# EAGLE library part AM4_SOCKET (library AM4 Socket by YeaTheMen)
Single Piece AM4 Socket Symbol. Every single one of the 1331 pins here in order Yours truly, YeaTheMen
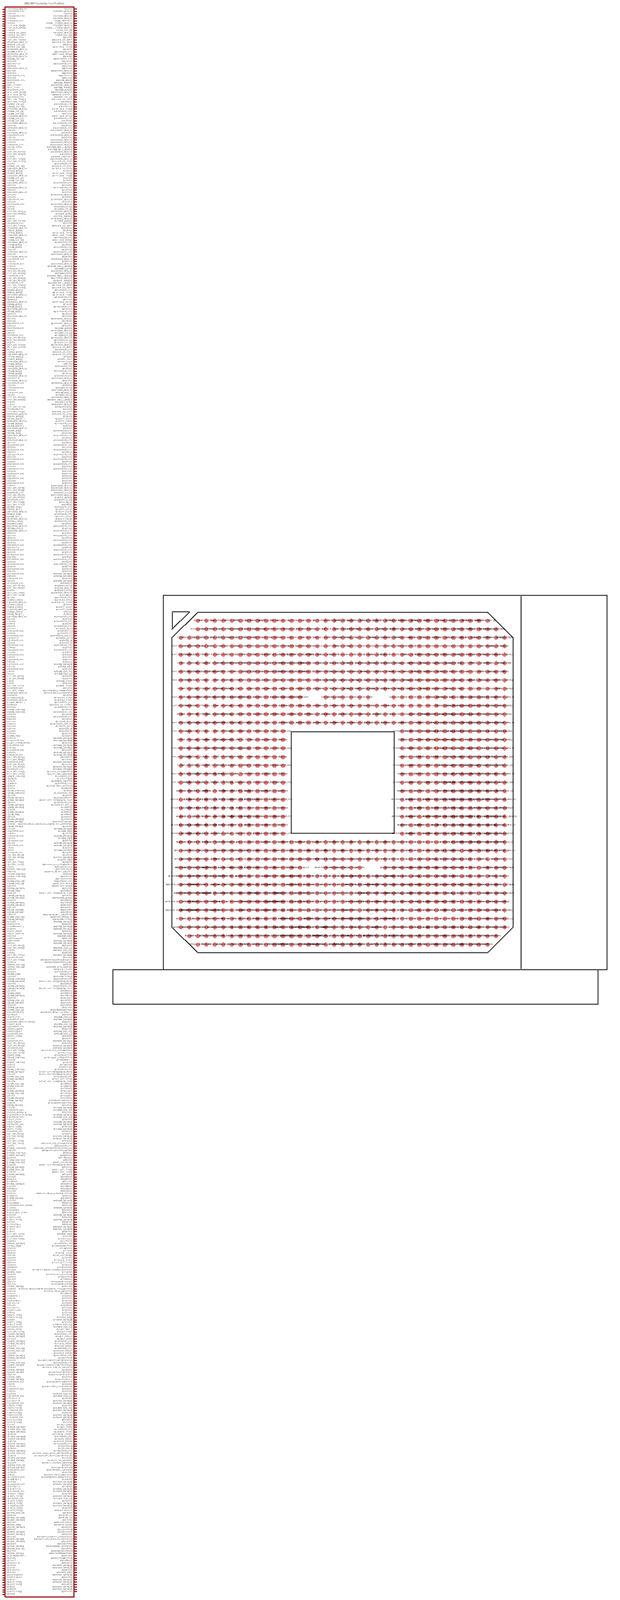
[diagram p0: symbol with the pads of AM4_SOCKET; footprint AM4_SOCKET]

Designator prefix -

## AM4_SOCKET  [AM4_SOCKET]
A3.VSS  A3.VSS  out
A4.DP0_TXN[2]  A4.DP0_TXN[2]
A5.RSVD  A5.RSVD  nc
A6.VSS  A6.VSS  out
A7.DP2_TXP[1]  A7.DP2_TXP[1]
A8.DP2_TXN[1]  A8.DP2_TXN[1]
A9.VSS  A9.VSS  out
A10.DP2_AUXP  A10.DP2_AUXP
A11.DP2_AUXN  A11.DP2_AUXN
A12.VSS  A12.VSS  out
A13.TEST11  A13.TEST11
A14.TDI  A14.TDI
A15.VSS  A15.VSS  out
A16.TEST41  A16.TEST41
A17.SVT  A17.SVT
A18.VSS  A18.VSS  out
A19.THERMTRIP_L  A19.THERMTRIP_L
A20.MB_DATA[4]  A20.MB_DATA[4]
A21.VSS  A21.VSS  out
A22.MB_DQS_L[0]  A22.MB_DQS_L[0]
A23.MB_DATA[6]  A23.MB_DATA[6]
A24.VSS  A24.VSS  out
A25.MB_DATA[12]  A25.MB_DATA[12]
A26.MB_DATA[8]  A26.MB_DATA[8]
A27.VSS  A27.VSS  out
A28.MB_DATA[14]  A28.MB_DATA[14]
A29.MB_DATA[10]  A29.MB_DATA[10]
A30.VSS  A30.VSS  out
A31.MB_DATA[16]  A31.MB_DATA[16]
A32.MB_DM[2]  A32.MB_DM[2]
A33.VSS  A33.VSS  out
A34.MB_DATA[23]  A34.MB_DATA[23]
A35.MB_DATA[28]  A35.MB_DATA[28]
A36.VSS  A36.VSS  out
A37.MB_DQS_L[3]  A37.MB_DQS_L[3]
AA1.VSS  AA1.VSS  out
AA2.USB_SS_1RXP  AA2.USB_SS_1RXP
AA3.USB_SS_1RXN  AA3.USB_SS_1RXN
AA4.VSS  AA4.VSS  out
AA5.P_HUB_TXP[1]  AA5.P_HUB_TXP[1]
AA6.VSS  AA6.VSS  out
AA7.VDDCR_CPU  AA7.VDDCR_CPU  pwr
AA8.P_HUB_RXN[1]  AA8.P_HUB_RXN[1]
AA9.VSS  AA9.VSS  out
AA10.VDDCR_CPU  AA10.VDDCR_CPU  pwr
AA11.VSS  AA11.VSS  out
AA12.VDDCR_CPU  AA12.VDDCR_CPU  pwr
AA13.VSS  AA13.VSS  out
AA27.VSS  AA27.VSS  out
AA28.VDDIO_MEM_S3  AA28.VDDIO_MEM_S3  pwr
AA29.VSS  AA29.VSS  out
AA30.TEST31  AA30.TEST31
AA31.VSS  AA31.VSS  out
AA32.MA_ADD[0]  AA32.MA_ADD[0]
AA33.MA_BANK[1]  AA33.MA_BANK[1]
AA34.VDDIO_MEM_S3  AA34.VDDIO_MEM_S3  pwr
AA35.MA_BANK[0]  AA35.MA_BANK[0]
AA36.MA_ADD[10]  AA36.MA_ADD[10]
AA37.VDDIO_MEM_S3  AA37.VDDIO_MEM_S3  pwr
AA38.MB_EVENT_L  AA38.MB_EVENT_L
AA39.MB_CLK_L[3]  AA39.MB_CLK_L[3]
AB1.USB_SS_1TXP  AB1.USB_SS_1TXP
AB2.RSVD  AB2.RSVD  nc
AB3.VDDCR_CPU  AB3.VDDCR_CPU  pwr
AB4.TEST10  AB4.TEST10
AB5.P_HUB_TXN[1]  AB5.P_HUB_TXN[1]
AB6.VDDCR_CPU  AB6.VDDCR_CPU  pwr
AB7.VSS  AB7.VSS  out
AB8.P_HUB_RXP[1]  AB8.P_HUB_RXP[1]
AB9.VDDCR_CPU  AB9.VDDCR_CPU  pwr
AB10.VSS  AB10.VSS  out
AB11.VDDCR_CPU  AB11.VDDCR_CPU  pwr
AB12.VSS  AB12.VSS  out
AB13.VDDCR_CPU  AB13.VDDCR_CPU  pwr
AB27.VDDIO_MEM_S3  AB27.VDDIO_MEM_S3  pwr
AB28.VSS  AB28.VSS  out
AB29.VDDIO_MEM_S3  AB29.VDDIO_MEM_S3  pwr
AB30.VSS  AB30.VSS  out
AB31.VDDIO_MEM_S3  AB31.VDDIO_MEM_S3  pwr
AB32.VDDIO_MEM_S3  AB32.VDDIO_MEM_S3  pwr
AB33.VDDIO_MEM_S3  AB33.VDDIO_MEM_S3  pwr
AB34.MA_RAS_L_ADD[16]  AB34.MA_RAS_L_ADD[16]
AB35.MA_WE_L_ADD[14]  AB35.MA_WE_L_ADD[14]
AB36.VDDIO_MEM_S3  AB36.VDDIO_MEM_S3  pwr
AB37.RSVD  AB37.RSVD  nc
AB38.MB_PARTOUT  AB38.MB_PARTOUT  out
AB39.VDDIO_MEM_S3  AB39.VDDIO_MEM_S3  pwr
AC1.USB_SS_1TXN  AC1.USB_SS_1TXN
AC2.VDDCR_CPU  AC2.VDDCR_CPU  pwr
AC3.USB_SS_2TXP  AC3.USB_SS_2TXP
AC4.USB_SS_2TXN  AC4.USB_SS_2TXN
AC5.VSS  AC5.VSS  out
AC6.P_HUB_TXP[2]  AC6.P_HUB_TXP[2]
AC7.P_HUB_TXN[2]  AC7.P_HUB_TXN[2]
AC8.VSS  AC8.VSS  out
AC9.VSS  AC9.VSS  out
AC10.VDDCR_CPU  AC10.VDDCR_CPU  pwr
AC11.VSS  AC11.VSS  out
AC12.VDDCR_CPU  AC12.VDDCR_CPU  pwr
AC13.VSS  AC13.VSS  out
AC27.VSS  AC27.VSS  out
AC28.VDDIO_MEM_S3  AC28.VDDIO_MEM_S3  pwr
AC29.VSS  AC29.VSS  out
AC30.VDDIO_MEM_S3  AC30.VDDIO_MEM_S3  pwr
AC31.VSS  AC31.VSS  out
AC32.VDDIO_MEM_S3  AC32.VDDIO_MEM_S3  pwr
AC33.MA0_CS_L[0]  AC33.MA0_CS_L[0]
AC34.MA1_CS_L[0]  AC34.MA1_CS_L[0]
AC35.VDDIO_MEM_S3  AC35.VDDIO_MEM_S3  pwr
AC36.MB_ADD[0]  AC36.MB_ADD[0]
AC37.MB_BANK[1]  AC37.MB_BANK[1]
AC38.VDDIO_MEM_S3  AC38.VDDIO_MEM_S3  pwr
AC39.MB_ADD[10]  AC39.MB_ADD[10]
AD1.VSS  AD1.VSS  out
AD2.USB_SS_3RXP  AD2.USB_SS_3RXP
AD3.RSVD  AD3.RSVD  nc
AD4.VSS  AD4.VSS  out
AD5.P_HUB_TXP[3]  AD5.P_HUB_TXP[3]
AD6.P_HUB_TXN[3]  AD6.P_HUB_TXN[3]
AD7.VDDCR_CPU  AD7.VDDCR_CPU  pwr
AD8.P_HUB_RXN[0]  AD8.P_HUB_RXN[0]
AD9.VDDCR_CPU  AD9.VDDCR_CPU  pwr
AD10.VSS  AD10.VSS  out
AD11.VDDCR_CPU  AD11.VDDCR_CPU  pwr
AD12.VSS  AD12.VSS  out
AD13.VDDCR_CPU  AD13.VDDCR_CPU  pwr
AD27.VDDIO_MEM_S3  AD27.VDDIO_MEM_S3  pwr
AD28.VSS  AD28.VSS  out
AD29.VDDIO_MEM_S3  AD29.VDDIO_MEM_S3  pwr
AD30.VSS  AD30.VSS  out
AD31.VDDIO_MEM_S3  AD31.VDDIO_MEM_S3  pwr
AD32.MA_CAS_L_ADD[15]  AD32.MA_CAS_L_ADD[15]
AD33.MA1_ODT[0]  AD33.MA1_ODT[0]
AD34.VDDIO_MEM_S3  AD34.VDDIO_MEM_S3  pwr
AD35.MA0_ODT[0]  AD35.MA0_ODT[0]
AD36.MB_RAS_L_ADD[16]  AD36.MB_RAS_L_ADD[16]
AD37.VDDIO_MEM_S3  AD37.VDDIO_MEM_S3  pwr
AD38.MB_BANK[0]  AD38.MB_BANK[0]
AD39.MB_WE_L_ADD[14]  AD39.MB_WE_L_ADD[14]
AE1.USB_SS_3RXP  AE1.USB_SS_3RXP
AE2.USB_SS_2RXN  AE2.USB_SS_2RXN
AE3.VDDCR_CPU  AE3.VDDCR_CPU  pwr
AE4.P_HUB_TXP[0]  AE4.P_HUB_TXP[0]
AE5.P_HUB_TXN[0]  AE5.P_HUB_TXN[0]
AE6.VDDCR_CPU  AE6.VDDCR_CPU  pwr
AE7.VSS  AE7.VSS  out
AE8.P_HUB_RXP[0]  AE8.P_HUB_RXP[0]
AE9.VSS  AE9.VSS  out
AE10.VDDCR_CPU  AE10.VDDCR_CPU  pwr
AE11.VSS  AE11.VSS  out
AE12.VDDCR_CPU  AE12.VDDCR_CPU  pwr
AE13.VSS  AE13.VSS  out
AE27.VSS  AE27.VSS  out
AE28.VDDIO_MEM_S3  AE28.VDDIO_MEM_S3  pwr
AE29.VSS  AE29.VSS  out
AE30.VDDIO_MEM_S3  AE30.VDDIO_MEM_S3  pwr
AE31.VSS  AE31.VSS  out
AE32.MA_ADD[13]  AE32.MA_ADD[13]
AE33.VDDIO_MEM_S3  AE33.VDDIO_MEM_S3  pwr
AE34.MA1_CS_L[1]  AE34.MA1_CS_L[1]
AE35.MA0_CS_L[1]  AE35.MA0_CS_L[1]
AE36.VDDIO_MEM_S3  AE36.VDDIO_MEM_S3  pwr
AE37.MB0_CS_L[0]  AE37.MB0_CS_L[0]
AE38.MB1_CS_L[0]  AE38.MB1_CS_L[0]
AE39.VDDIO_MEM_S3  AE39.VDDIO_MEM_S3  pwr
AF1.USB_SS_3RXN  AF1.USB_SS_3RXN
AF2.VDDCR_CPU  AF2.VDDCR_CPU  pwr
AF3.USB_SS_0TXP  AF3.USB_SS_0TXP
AF4.USB_SS_0TXN  AF4.USB_SS_0TXN
AF5.VSS  AF5.VSS  out
AF6.GFX_CLKP  AF6.GFX_CLKP
AF7.GFX_CLKN  AF7.GFX_CLKN
AF8.VSS  AF8.VSS  out
AF9.VDDCR_CPU  AF9.VDDCR_CPU  pwr
AF10.VSS  AF10.VSS  out
AF11.VDDCR_CPU  AF11.VDDCR_CPU  pwr
AF12.VSS  AF12.VSS  out
AF13.VDDCR_CPU  AF13.VDDCR_CPU  pwr
AF27.VDDIO_MEM_S3  AF27.VDDIO_MEM_S3  pwr
AF28.VSS  AF28.VSS  out
AF29.VDDIO_MEM_S3  AF29.VDDIO_MEM_S3  pwr
AF30.VSS  AF30.VSS  out
AF31.MA0_ODT[1]  AF31.MA0_ODT[1]
AF32.VDDIO_MEM_S3  AF32.VDDIO_MEM_S3  pwr
AF33.MA_ADD_17  AF33.MA_ADD_17
AF34.MA1_ODT[1]  AF34.MA1_ODT[1]
AF35.VDDIO_MEM_S3  AF35.VDDIO_MEM_S3  pwr
AF36.MB_CAS_L_ADD[15]  AF36.MB_CAS_L_ADD[15]
AF37.MB1_ODT[0]  AF37.MB1_ODT[0]
AF38.VDDIO_MEM_S3  AF38.VDDIO_MEM_S3  pwr
AF39.MB0_ODT[0]  AF39.MB0_ODT[0]
AG1.VSS  AG1.VSS  out
AG2.USB_SS_3TXP  AG2.USB_SS_3TXP
AG3.USB_SS_3TXN  AG3.USB_SS_3TXN
AG4.VSS  AG4.VSS  out
AG5.GPP_CLK0P  AG5.GPP_CLK0P
AG6.GPP_CLK0N  AG6.GPP_CLK0N
AG7.VDDCR_CPU  AG7.VDDCR_CPU  pwr
AG8.VSS  AG8.VSS  out
AG9.VSS  AG9.VSS  out
AG10.VDDCR_CPU  AG10.VDDCR_CPU  pwr
AG11.VSS  AG11.VSS  out
AG12.VDDCR_CPU  AG12.VDDCR_CPU  pwr
AG13.VSS  AG13.VSS  out
AG14.VDDCR_CPU  AG14.VDDCR_CPU  pwr
AG15.VSS  AG15.VSS  out
AG16.VDDCR_CPU  AG16.VDDCR_CPU  pwr
AG17.VSS  AG17.VSS  out
AG18.VDDCR_CPU  AG18.VDDCR_CPU  pwr
AG19.VSS  AG19.VSS  out
AG20.VDDCR_CPU  AG20.VDDCR_CPU  pwr
AG21.VSS  AG21.VSS  out
AG22.VDDCR_CPU  AG22.VDDCR_CPU  pwr
AG23.VSS  AG23.VSS  out
AG24.VDDCR_CPU  AG24.VDDCR_CPU  pwr
AG25.VSS  AG25.VSS  out
AG26.VDDCR_CPU  AG26.VDDCR_CPU  pwr
AG27.VSS  AG27.VSS  out
AG28.VSS  AG28.VSS  out
AG29.VSS  AG29.VSS  out
AG30.VSS  AG30.VSS  out
AG31.VSS  AG31.VSS  out
AG32.VSS  AG32.VSS  out
AG33.VDDIO_MEM_S3  AG33.VDDIO_MEM_S3  pwr
AG34.VDDIO_MEM_S3  AG34.VDDIO_MEM_S3  pwr
AG35.VDDIO_MEM_S3  AG35.VDDIO_MEM_S3  pwr
AG36.MB1_CS_L[1]  AG36.MB1_CS_L[1]
AG37.VDDIO_MEM_S3  AG37.VDDIO_MEM_S3  pwr
AG38.MB_ADD[13]  AG38.MB_ADD[13]
AG39.MB0_CS_L[1]  AG39.MB0_CS_L[1]
AH1.X48M_X2  AH1.X48M_X2
AH2.RSVD  AH2.RSVD  nc
AH3.VDDCR_CPU  AH3.VDDCR_CPU  pwr
AH4.GPP_CLK1P  AH4.GPP_CLK1P
AH5.GPP_CLK1N  AH5.GPP_CLK1N
AH6.VDDCR_CPU  AH6.VDDCR_CPU  pwr
AH7.GPP_CLK2P  AH7.GPP_CLK2P
AH8.GPP_CLK2N  AH8.GPP_CLK2N
AH9.VDDCR_CPU  AH9.VDDCR_CPU  pwr
AH10.VSS  AH10.VSS  out
AH11.VDDCR_CPU  AH11.VDDCR_CPU  pwr
AH12.VSS  AH12.VSS  out
AH13.VDDCR_CPU  AH13.VDDCR_CPU  pwr
AH14.VSS  AH14.VSS  out
AH15.VDDCR_CPU  AH15.VDDCR_CPU  pwr
AH16.VSS  AH16.VSS  out
AH17.VDDCR_CPU  AH17.VDDCR_CPU  pwr
AH18.VSS  AH18.VSS  out
AH19.VDDCR_CPU  AH19.VDDCR_CPU  pwr
AH20.VSS  AH20.VSS  out
AH21.VDDCR_CPU  AH21.VDDCR_CPU  pwr
AH22.VSS  AH22.VSS  out
AH23.VDDCR_CPU  AH23.VDDCR_CPU  pwr
AH24.VSS  AH24.VSS  out
AH25.VDDCR_CPU  AH25.VDDCR_CPU  pwr
AH26.VSS  AH26.VSS  out
AH27.VDDCR_CPU  AH27.VDDCR_CPU  pwr
AH28.VSS  AH28.VSS  out
AH29.VSS  AH29.VSS  out
AH30.VSS  AH30.VSS  out
AH31.MA_DATA[36]  AH31.MA_DATA[36]
AH32.MA_DATA[37]  AH32.MA_DATA[37]
AH33.VSS  AH33.VSS  out
AH34.MA_DATA[32]  AH34.MA_DATA[32]
AH35.RSVD  AH35.RSVD  nc
AH36.MB0_ODT[1]  AH36.MB0_ODT[1]
AH37.MB_ADD_17  AH37.MB_ADD_17
AH38.MB1_ODT[1]  AH38.MB1_ODT[1]
AH39.VDDIO_MEM_S3  AH39.VDDIO_MEM_S3  pwr
AJ1.X48M_X1  AJ1.X48M_X1
AJ2.VDDCR_CPU  AJ2.VDDCR_CPU  pwr
AJ3.USB0_ZVSS  AJ3.USB0_ZVSS  out
AJ4.USB_SS_ZVSS  AJ4.USB_SS_ZVSS  out
AJ5.VSS  AJ5.VSS  out
AJ6.GPP_CLK3P  AJ6.GPP_CLK3P
AJ7.GPP_CLK3N  AJ7.GPP_CLK3N
AJ8.VSS  AJ8.VSS  out
AJ9.VSS  AJ9.VSS  out
AJ10.VDDCR_CPU  AJ10.VDDCR_CPU  pwr
AJ11.VSS  AJ11.VSS  out
AJ12.VDDCR_CPU  AJ12.VDDCR_CPU  pwr
AJ13.VSS  AJ13.VSS  out
AJ14.VDDCR_CPU  AJ14.VDDCR_CPU  pwr
AJ15.VDD_18_S5  AJ15.VDD_18_S5  pwr
AJ16.VDDP_S5  AJ16.VDDP_S5  pwr
AJ17.VDDP_S5  AJ17.VDDP_S5  pwr
AJ18.VDDCR_SOC_S5  AJ18.VDDCR_SOC_S5  pwr
AJ19.VDD_33_S5  AJ19.VDD_33_S5  pwr
AJ20.VDD_18  AJ20.VDD_18  pwr
AJ21.VDD_33  AJ21.VDD_33  pwr
AJ22.VDDCR_CPU  AJ22.VDDCR_CPU  pwr
AJ23.VSS  AJ23.VSS  out
AJ24.VDDCR_CPU  AJ24.VDDCR_CPU  pwr
AJ25.VSS  AJ25.VSS  out
AJ26.VSS  AJ26.VSS  out
AJ27.VSS  AJ27.VSS  out
AJ28.VSS  AJ28.VSS  out
AJ29.VSS  AJ29.VSS  out
AJ30.MA_DATA[33]  AJ30.MA_DATA[33]
AJ31.MA_DM[4]  AJ31.MA_DM[4]
AJ32.VSS  AJ32.VSS  out
AJ33.MA_DQS_H[4]  AJ33.MA_DQS_H[4]
AJ34.MA_DQS_L[4]  AJ34.MA_DQS_L[4]
AJ35.VSS  AJ35.VSS  out
AJ36.VSS  AJ36.VSS  out
AJ37.MA_ZVSS  AJ37.MA_ZVSS  out
AJ38.VSS  AJ38.VSS  out
AJ39.MB_ZVSS  AJ39.MB_ZVSS  out
AK1.VSS  AK1.VSS  out
AK2.SDA1/I2C3_SDA/AGPIO20  AK2.SDA1/I2C3_SDA/AGPIO20
AK3.SCL1/I2C3_SCL/AGPIO19  AK3.SCL1/I2C3_SCL/AGPIO19
AK4.VSS  AK4.VSS  out
AK5.USB3_ZVSS  AK5.USB3_ZVSS  out
AK6.USB2_ZVSS  AK6.USB2_ZVSS  out
AK7.VDDCR_CPU  AK7.VDDCR_CPU  pwr
AK8.USB_SS_ZVDDP  AK8.USB_SS_ZVDDP  pwr
AK9.VDDCR_CPU  AK9.VDDCR_CPU  pwr
AK10.VSS  AK10.VSS  out
AK11.VDDCR_CPU  AK11.VDDCR_CPU  pwr
AK12.VSS  AK12.VSS  out
AK13.VDDCR_CPU  AK13.VDDCR_CPU  pwr
AK14.VSS  AK14.VSS  out
AK15.VDD_18_S5  AK15.VDD_18_S5  pwr
AK18.VDDCR_SOC_S5  AK18.VDDCR_SOC_S5  pwr
AK19.VDD_33_S5  AK19.VDD_33_S5  pwr
AK20.VDD_18  AK20.VDD_18  pwr
AK21.VDD_33  AK21.VDD_33  pwr
AK22.VSS  AK22.VSS  out
AK25.VSS  AK25.VSS  out
AK26.MA_DATA[57]  AK26.MA_DATA[57]
AK27.MA_DATA[56]  AK27.MA_DATA[56]
AK28.VSS  AK28.VSS  out
AK29.MA_DATA[49]  AK29.MA_DATA[49]
AK30.MA_DATA[34]  AK30.MA_DATA[34]
AK31.VSS  AK31.VSS  out
AK32.MA_DATA[39]  AK32.MA_DATA[39]
AK33.MA_DATA[38]  AK33.MA_DATA[38]
AK34.RSVD  AK34.RSVD  nc
AK35.VSS  AK35.VSS  out
AK36.MB_DATA[37]  AK36.MB_DATA[37]
AK37.VSS  AK37.VSS  out
AK38.MB_DATA[36]  AK38.MB_DATA[36]
AK39.MB_DATA[32]  AK39.MB_DATA[32]
AL1.USB_OC0_L/AGPIO16  AL1.USB_OC0_L/AGPIO16
AL2.LPC_PME_L/AGPIO22  AL2.LPC_PME_L/AGPIO22
AL3.VDDCR_CPU  AL3.VDDCR_CPU  pwr
AL4.TEST46[13]  AL4.TEST46[13]
AL5.WAKE_L/AGPIO2  AL5.WAKE_L/AGPIO2
AL6.VDDCR_CPU  AL6.VDDCR_CPU  pwr
AL7.PCIE_RST_L/EGPIO26  AL7.PCIE_RST_L/EGPIO26
AL8.AM4R1  AL8.AM4R1
AL9.VSS  AL9.VSS  out
AL10.VDDCR_CPU  AL10.VDDCR_CPU  pwr
AL11.VSS  AL11.VSS  out
AL12.VDDCR_CPU  AL12.VDDCR_CPU  pwr
AL13.P_GPP_TXP[2]/SATA_TX0P  AL13.P_GPP_TXP[2]/SATA_TX0P
AL14.VDDCR_CPU  AL14.VDDCR_CPU  pwr
AL15.VDDBT_RTC_G  AL15.VDDBT_RTC_G  pwr
AL16.RSVD  AL16.RSVD  nc
AL17.RSVD  AL17.RSVD  nc
AL18.RSVD  AL18.RSVD  nc
AL19.RSVD  AL19.RSVD  nc
AL20.RSVD  AL20.RSVD  nc
AL21.RSVD  AL21.RSVD  nc
AL22.VDDP_SENSE  AL22.VDDP_SENSE  pwr
AL23.CLK_REQ3_L/SATA_IS1_L/SATA_ZP1_L/EGPIO131  AL23.CLK_REQ3_L/SATA_IS1_L/SATA_ZP1_L/EGPIO131
AL24.VSS  AL24.VSS  out
AL25.MA_DATA[62]  AL25.MA_DATA[62]
AL26.MA_DM[7]  AL26.MA_DM[7]
AL27.VSS  AL27.VSS  out
AL28.MA_DATA[51]  AL28.MA_DATA[51]
AL29.MA_DM[6]  AL29.MA_DM[6]
AL30.VSS  AL30.VSS  out
AL31.MA_DATA[45]  AL31.MA_DATA[45]
AL32.MA_DATA[44]  AL32.MA_DATA[44]
AL33.VSS  AL33.VSS  out
AL34.MA_DATA[35]  AL34.MA_DATA[35]
AL35.VSS  AL35.VSS  out
AL36.VSS  AL36.VSS  out
AL37.MB_DATA[33]  AL37.MB_DATA[33]
AL38.MB_DM[4]  AL38.MB_DM[4]
AL39.VSS  AL39.VSS  out
AM1.USB_OC1_L/TDI/AGPIO17  AM1.USB_OC1_L/TDI/AGPIO17
AM2.VDDCR_CPU  AM2.VDDCR_CPU  pwr
AM3.PWR_GOOD  AM3.PWR_GOOD
AM4.SYS_RESET_L/AGPIO1  AM4.SYS_RESET_L/AGPIO1
AM5.VSS  AM5.VSS  out
AM6.TEST0  AM6.TEST0
AM7.TEST1/TMS  AM7.TEST1/TMS
AM8.VDDCR_CPU  AM8.VDDCR_CPU  pwr
AM9.P_GPP_RXP[1]  AM9.P_GPP_RXP[1]
AM10.P_GPP_RXN[1]  AM10.P_GPP_RXN[1]
AM11.VSS  AM11.VSS  out
AM12.RSVD  AM12.RSVD  nc
AM13.P_GPP_TXN[2]/SATA_TX0N  AM13.P_GPP_TXN[2]/SATA_TX0N
AM14.VSS  AM14.VSS  out
AM15.VDDIO_AUDIO  AM15.VDDIO_AUDIO  pwr
AM16.RSVD  AM16.RSVD  nc
AM17.RSVD  AM17.RSVD  nc
AM18.VDDP  AM18.VDDP  pwr
AM19.VDDP  AM19.VDDP  pwr
AM20.VDDP  AM20.VDDP  pwr
AM21.RSVD  AM21.RSVD  nc
AM22.SATA_ACT_L/AGPIO130  AM22.SATA_ACT_L/AGPIO130
AM23.VSS_SENSE_B  AM23.VSS_SENSE_B
AM24.CORETYPE[0]  AM24.CORETYPE[0]
AM25.MA_DATA[63]  AM25.MA_DATA[63]
AM26.VSS  AM26.VSS  out
AM27.MA_DATA[61]  AM27.MA_DATA[61]
AM28.MA_DATA[50]  AM28.MA_DATA[50]
AM29.VSS  AM29.VSS  out
AM30.MA_DATA[52]  AM30.MA_DATA[52]
AM31.MA_DM[5]  AM31.MA_DM[5]
AM32.VSS  AM32.VSS  out
AM33.MA_DATA[41]  AM33.MA_DATA[41]
AM34.MA_DATA[40]  AM34.MA_DATA[40]
AM35.VSS  AM35.VSS  out
AM36.MB_DQS_L[4]  AM36.MB_DQS_L[4]
AM37.MB_DQS_H[4]  AM37.MB_DQS_H[4]
AM38.VSS  AM38.VSS  out
AM39.MB_DATA[38]  AM39.MB_DATA[38]
AN1.VSS  AN1.VSS  out
AN2.AGPIO9/SGPIO0_DATAOUT  AN2.AGPIO9/SGPIO0_DATAOUT  out
AN3.AGPIO23/SGPIO0_LOAD  AN3.AGPIO23/SGPIO0_LOAD
AN4.VSS  AN4.VSS  out
AN5.PWR_BTN_L/AGPIO0  AN5.PWR_BTN_L/AGPIO0
AN6.USB1_ZVSS  AN6.USB1_ZVSS  out
AN7.VDDCR_CPU  AN7.VDDCR_CPU  pwr
AN8.AGPIO6  AN8.AGPIO6
AN9.CORETYPE[1]  AN9.CORETYPE[1]
AN10.VDDCR_CPU  AN10.VDDCR_CPU  pwr
AN11.P_GPP_RXN[3]/SATA_RX1N  AN11.P_GPP_RXN[3]/SATA_RX1N
AN12.RSVD  AN12.RSVD  nc
AN13.VDDCR_CPU  AN13.VDDCR_CPU  pwr
AN14.P_GPP_TXP[3]/SATA_TX1P  AN14.P_GPP_TXP[3]/SATA_TX1P
AN15.RSVD  AN15.RSVD  nc
AN16.RSVD  AN16.RSVD  nc
AN17.RSVD  AN17.RSVD  nc
AN18.VDDP  AN18.VDDP  pwr
AN19.VDDP  AN19.VDDP  pwr
AN20.VDDP  AN20.VDDP  pwr
AN21.RSVD  AN21.RSVD  nc
AN22.VSS  AN22.VSS  out
AN23.FANIN0/AGPIO84  AN23.FANIN0/AGPIO84  in
AN24.ESPI_RESET_L/KBRST_L  AN24.ESPI_RESET_L/KBRST_L
AN25.VSS  AN25.VSS  out
AN26.MA_DQS_L[7]  AN26.MA_DQS_L[7]
AN27.MA_DATA[60]  AN27.MA_DATA[60]
AN28.VSS  AN28.VSS  out
AN29.MA_DQS_L[6]  AN29.MA_DQS_L[6]
AN30.MA_DATA[53]  AN30.MA_DATA[53]
AN31.VSS  AN31.VSS  out
AN32.MA_DQS_H[5]  AN32.MA_DQS_H[5]
AN33.MA_DQS_L[5]  AN33.MA_DQS_L[5]
AN34.VSS  AN34.VSS  out
AN35.VSS  AN35.VSS  out
AN36.MB_DATA[34]  AN36.MB_DATA[34]
AN37.VSS  AN37.VSS  out
AN38.MB_DATA[39]  AN38.MB_DATA[39]
AN39.MB_DATA[35]  AN39.MB_DATA[35]
AP1.USB_OC3_L/TDO/AGPIO24  AP1.USB_OC3_L/TDO/AGPIO24
AP2.SLP_S5_L  AP2.SLP_S5_L
AP3.VDDCR_CPU  AP3.VDDCR_CPU  pwr
AP4.S5_MUX_CTRL/EGPIO42  AP4.S5_MUX_CTRL/EGPIO42
AP5.RSMRST_L  AP5.RSMRST_L
AP6.VSS  AP6.VSS  out
AP7.AGPIO8  AP7.AGPIO8
AP8.RTCCLK  AP8.RTCCLK
AP9.VDDCR_CPU  AP9.VDDCR_CPU  pwr
AP10.P_GPP_RXN[2]/SATA_RX0N  AP10.P_GPP_RXN[2]/SATA_RX0N
AP11.P_GPP_RXP[3]/SATA_RX1P  AP11.P_GPP_RXP[3]/SATA_RX1P
AP12.VDDCR_CPU  AP12.VDDCR_CPU  pwr
AP13.P_GPP_TXP[1]  AP13.P_GPP_TXP[1]
AP14.P_GPP_TXN[3]/SATA_TX1N  AP14.P_GPP_TXN[3]/SATA_TX1N
AP15.RSVD  AP15.RSVD  nc
AP16.RSVD  AP16.RSVD  nc
AP17.RSVD  AP17.RSVD  nc
AP18.VDDP  AP18.VDDP  pwr
AP19.VDDP  AP19.VDDP  pwr
AP20.VDDP  AP20.VDDP  pwr
AP21.RSVD  AP21.RSVD  nc
AP22.AGPIO5/DEVSLP0  AP22.AGPIO5/DEVSLP0
AP23.FANOUT0/AGPIO85  AP23.FANOUT0/AGPIO85  out
AP24.VSS  AP24.VSS  out
AP25.MA_DATA[58]  AP25.MA_DATA[58]
AP26.MA_DQS_H[7]  AP26.MA_DQS_H[7]
AP27.VSS  AP27.VSS  out
AP28.MA_DATA[54]  AP28.MA_DATA[54]
AP29.MA_DQS_H[6]  AP29.MA_DQS_H[6]
AP30.VSS  AP30.VSS  out
AP31.MA_DATA[42]  AP31.MA_DATA[42]
AP32.MA_DATA[47]  AP32.MA_DATA[47]
AP33.VSS  AP33.VSS  out
AP34.MA_DATA[46]  AP34.MA_DATA[46]
AP35.VSS  AP35.VSS  out
AP36.VSS  AP36.VSS  out
AP37.MB_DATA[44]  AP37.MB_DATA[44]
AP38.MB_DATA[45]  AP38.MB_DATA[45]
AP39.VSS  AP39.VSS  out
AR1.USB_OC2_L/TCK/AGPIO18  AR1.USB_OC2_L/TCK/AGPIO18
AR2.VDDCR_CPU  AR2.VDDCR_CPU  pwr
AR3.S0A3_GPIO/AGPIO10/SGPIO0_CLK  AR3.S0A3_GPIO/AGPIO10/SGPIO0_CLK
AR4.AGPIO40/SGPIO0_DATAIN  AR4.AGPIO40/SGPIO0_DATAIN  in
AR5.VSS  AR5.VSS  out
AR6.AGPIO4  AR6.AGPIO4
AR7.48M_OSC  AR7.48M_OSC
AR8.VSS  AR8.VSS  out
AR9.P_GPP_RXP[0]  AR9.P_GPP_RXP[0]
AR10.P_GPP_RXP[2]/SATA_RX0P  AR10.P_GPP_RXP[2]/SATA_RX0P
AR11.VSS  AR11.VSS  out
AR12.P_GPP_TXN[0]  AR12.P_GPP_TXN[0]
AR13.P_GPP_TXN[1]  AR13.P_GPP_TXN[1]
AR14.VSS  AR14.VSS  out
AR15.RSVD  AR15.RSVD  nc
AR16.RSVD  AR16.RSVD  nc
AR17.VSS  AR17.VSS  out
AR18.RSVD  AR18.RSVD  nc
AR19.RSVD  AR19.RSVD  nc
AR20.RSVD  AR20.RSVD  nc
AR21.RSVD  AR21.RSVD  nc
AR22.CLK_REQG_L/OSCIN/EGPIO132  AR22.CLK_REQG_L/OSCIN/EGPIO132  in
AR23.VSS  AR23.VSS  out
AR24.RSVD  AR24.RSVD  nc
AR25.MA_DATA[59]  AR25.MA_DATA[59]
AR26.VSS  AR26.VSS  out
AR27.VSS  AR27.VSS  out
AR28.MA_DATA[55]  AR28.MA_DATA[55]
AR29.VSS  AR29.VSS  out
AR30.VSS  AR30.VSS  out
AR31.MA_DATA[48]  AR31.MA_DATA[48]
AR32.VSS  AR32.VSS  out
AR33.MA_DATA[43]  AR33.MA_DATA[43]
AR34.VSS  AR34.VSS  out
AR35.VSS  AR35.VSS  out
AR36.MB_DATA[40]  AR36.MB_DATA[40]
AR37.MB_DATA[41]  AR37.MB_DATA[41]
AR38.VSS  AR38.VSS  out
AR39.MB_DM[5]  AR39.MB_DM[5]
AT1.VSS  AT1.VSS  out
AT2.SLP_S3_L  AT2.SLP_S3_L
AT3.TEST2  AT3.TEST2
AT4.VDDCR_CPU  AT4.VDDCR_CPU  pwr
AT5.BLINK/AGPIO11  AT5.BLINK/AGPIO11  in
AT6.AGPIO3  AT6.AGPIO3
AT7.VSS  AT7.VSS  out
AT8.P0B_ZVSS  AT8.P0B_ZVSS  out
AT9.P_GPP_RXN[0]  AT9.P_GPP_RXN[0]
AT10.VSS  AT10.VSS  out
AT11.USB_ZVSS  AT11.USB_ZVSS  out
AT12.P_GPP_TXP[0]  AT12.P_GPP_TXP[0]
AT13.VSS  AT13.VSS  out
AT14.EGPIO100  AT14.EGPIO100
AT15.ESPI_ALERT_L/LDRQ0_L/EGPIO108  AT15.ESPI_ALERT_L/LDRQ0_L/EGPIO108
AT16.VSS  AT16.VSS  out
AT17.SPI_CS1_L/EGPIO118  AT17.SPI_CS1_L/EGPIO118
AT18.EGPIO70  AT18.EGPIO70
AT19.RSVD  AT19.RSVD  nc
AT20.LAD3/EGPIO107  AT20.LAD3/EGPIO107
AT21.LAD2/EGPIO106  AT21.LAD2/EGPIO106
AT22.VSS  AT22.VSS  out
AT23.CLK_REQ0_L/SATA_IS0_L/SATA_ZP0_L/AGPIO92  AT23.CLK_REQ0_L/SATA_IS0_L/SATA_ZP0_L/AGPIO92
AT24.CLK_REQ2_L/AGPIO116  AT24.CLK_REQ2_L/AGPIO116
AT25.RSVD  AT25.RSVD  nc
AT26.VSS  AT26.VSS  out
AT27.VSS  AT27.VSS  out
AT28.VSS  AT28.VSS  out
AT29.VSS  AT29.VSS  out
AT30.RSVD  AT30.RSVD  nc
AT31.VSS  AT31.VSS  out
AT32.VSS  AT32.VSS  out
AT33.VSS  AT33.VSS  out
AT34.VSS  AT34.VSS  out
AT35.MB_DM[6]  AT35.MB_DM[6]
AT36.MB_DATA[46]  AT36.MB_DATA[46]
AT37.VSS  AT37.VSS  out
AT38.MB_DQS_H[5]  AT38.MB_DQS_H[5]
AT39.MB_DQS_L[5]  AT39.MB_DQS_L[5]
AU1.AZ_RST_L  AU1.AZ_RST_L
AU2.AZ_SYNC  AU2.AZ_SYNC
AU3.VDDCR_CPU  AU3.VDDCR_CPU  pwr
AU4.AZ_SDOUT  AU4.AZ_SDOUT  out
AU5.AZ_SDIN1  AU5.AZ_SDIN1  in
AU6.VDDCR_CPU  AU6.VDDCR_CPU  pwr
AU7.USB_HSD0P  AU7.USB_HSD0P
AU8.USB_HSD0N  AU8.USB_HSD0N
AU9.VDDCR_CPU  AU9.VDDCR_CPU  pwr
AU10.USB_HSD2P  AU10.USB_HSD2P
AU11.USB_HSD2N  AU11.USB_HSD2N
AU12.VDDCR_CPU  AU12.VDDCR_CPU  pwr
AU13.EGPIO98  AU13.EGPIO98
AU14.SPI_DI/ESPI_DAT1/EGPIO120  AU14.SPI_DI/ESPI_DAT1/EGPIO120
AU15.VDDCR_CPU  AU15.VDDCR_CPU  pwr
AU16.SPI_DO/ESPI_DAT0/EGPIO121  AU16.SPI_DO/ESPI_DAT0/EGPIO121
AU17.SPI_TPM_CS_L/AGPIO76  AU17.SPI_TPM_CS_L/AGPIO76
AU18.VSS  AU18.VSS  out
AU19.LPCCLK1/EGPIO75  AU19.LPCCLK1/EGPIO75
AU20.LPCCLK0/EGPIO74  AU20.LPCCLK0/EGPIO74
AU21.VSS  AU21.VSS  out
AU22.LPC_RST_L  AU22.LPC_RST_L
AU23.GENINT2_L/AGPIO90  AU23.GENINT2_L/AGPIO90  in
AU24.VSS  AU24.VSS  out
AU25.SCL0/I2C2_SCL/EGPIO113  AU25.SCL0/I2C2_SCL/EGPIO113
AU26.VSS  AU26.VSS  out
AU27.VSS  AU27.VSS  out
AU28.MB_DQS_H[7]  AU28.MB_DQS_H[7]
AU29.MB_DQS_L[7]  AU29.MB_DQS_L[7]
AU30.VSS  AU30.VSS  out
AU31.MB_DATA[61]  AU31.MB_DATA[61]
AU32.MB_DATA[51]  AU32.MB_DATA[51]
AU33.VSS  AU33.VSS  out
AU34.MB_DQS_H[6]  AU34.MB_DQS_H[6]
AU35.MB_DATA[49]  AU35.MB_DATA[49]
AU36.VSS  AU36.VSS  out
AU37.MB_DATA[42]  AU37.MB_DATA[42]
AU38.MB_DATA[47]  AU38.MB_DATA[47]
AU39.VSS  AU39.VSS  out
AV2.VSS  AV2.VSS  out
AV3.AZ_SDIN0  AV3.AZ_SDIN0  in
AV4.AZ_SDIN2  AV4.AZ_SDIN2  in
AV5.VDDCR_CPU  AV5.VDDCR_CPU  pwr
AV6.SATA_ZVSS  AV6.SATA_ZVSS  out
AV7.SATA_ZVDDP  AV7.SATA_ZVDDP  pwr
AV8.VDDCR_CPU  AV8.VDDCR_CPU  pwr
AV9.USB_HSD3P  AV9.USB_HSD3P
AV10.USB_HSD3N  AV10.USB_HSD3N
AV11.VDDCR_CPU  AV11.VDDCR_CPU  pwr
AV12.EGPIO96  AV12.EGPIO96
AV13.EGPIO99  AV13.EGPIO99
AV14.VDDCR_CPU  AV14.VDDCR_CPU  pwr
AV15.SPI_HOLD_L/ESPI_DAT3/EGPIO133  AV15.SPI_HOLD_L/ESPI_DAT3/EGPIO133
AV16.SPI_WP_L/ESPI_DAT2/EGPIO122  AV16.SPI_WP_L/ESPI_DAT2/EGPIO122
AV17.VSS  AV17.VSS  out
AV18.LPC_PD_L/AGPIO21  AV18.LPC_PD_L/AGPIO21
AV19.LPC_CLKRUN_L/AGPIO88  AV19.LPC_CLKRUN_L/AGPIO88
AV20.VSS  AV20.VSS  out
AV21.LAD1/EGPIO105  AV21.LAD1/EGPIO105
AV22.GENINT1_L/AGPIO89  AV22.GENINT1_L/AGPIO89  in
AV23.VSS  AV23.VSS  out
AV24.CLK_REQ1_L/AGPIO115  AV24.CLK_REQ1_L/AGPIO115
AV25.SDA0/I2C2_SDA/EGPIO114  AV25.SDA0/I2C2_SDA/EGPIO114
AV26.VSS  AV26.VSS  out
AV27.MB_DATA[63]  AV27.MB_DATA[63]
AV28.MB_DATA[62]  AV28.MB_DATA[62]
AV29.VSS  AV29.VSS  out
AV30.MB_DATA[57]  AV30.MB_DATA[57]
AV31.MB_DATA[60]  AV31.MB_DATA[60]
AV32.VSS  AV32.VSS  out
AV33.MB_DATA[55]  AV33.MB_DATA[55]
AV34.MB_DQS_L[6]  AV34.MB_DQS_L[6]
AV35.VSS  AV35.VSS  out
AV36.MB_DATA[52]  AV36.MB_DATA[52]
AV37.MB_DATA[43]  AV37.MB_DATA[43]
AV38.VSS  AV38.VSS  out
AW3.AZ_BITCLK  AW3.AZ_BITCLK
AW4.VSS  AW4.VSS  out
AW5.X32K_X1  AW5.X32K_X1
AW6.X32K_X2  AW6.X32K_X2
AW7.VSS  AW7.VSS  out
AW8.USB_HSD1P  AW8.USB_HSD1P
AW9.USB_HSD1N  AW9.USB_HSD1N
AW10.VSS  AW10.VSS  out
AW11.EGPIO95  AW11.EGPIO95
AW12.EGPIO97  AW12.EGPIO97
AW13.VSS  AW13.VSS  out
AW14.SPI_CLK/ESPI_CLK/EGPIO117  AW14.SPI_CLK/ESPI_CLK/EGPIO117
AW15.SPI_CS2_L/ESPI_CS_L/EGPIO119  AW15.SPI_CS2_L/ESPI_CS_L/EGPIO119
AW16.VSS  AW16.VSS  out
AW17.AGPIO86  AW17.AGPIO86
AW18.LFRAME_L/EGPIO109  AW18.LFRAME_L/EGPIO109
AW19.VSS  AW19.VSS  out
AW20.LAD0/EGPIO104  AW20.LAD0/EGPIO104
AW21.SERIRQ/AGPIO87  AW21.SERIRQ/AGPIO87
AW22.VSS  AW22.VSS  out
AW23.SPKR/AGPIO91  AW23.SPKR/AGPIO91
AW24.RSVD  AW24.RSVD  nc
AW25.VSS  AW25.VSS  out
AW26.MB_DATA[59]  AW26.MB_DATA[59]
AW27.MB_DATA[58]  AW27.MB_DATA[58]
AW28.VSS  AW28.VSS  out
AW29.MB_DM[7]  AW29.MB_DM[7]
AW30.MB_DATA[56]  AW30.MB_DATA[56]
AW31.VSS  AW31.VSS  out
AW32.MB_DATA[50]  AW32.MB_DATA[50]
AW33.MB_DATA[54]  AW33.MB_DATA[54]
AW34.VSS  AW34.VSS  out
AW35.MB_DATA[48]  AW35.MB_DATA[48]
AW36.MB_DATA[53]  AW36.MB_DATA[53]
AW37.VSS  AW37.VSS  out
B3.DP0_TXN[1]  B3.DP0_TXN[1]
B4.DP0_TXP[2]  B4.DP0_TXP[2]
B5.VDDCR_SOC  B5.VDDCR_SOC  pwr
B6.DP2_TXP[0]  B6.DP2_TXP[0]
B7.DP2_TXN[0]  B7.DP2_TXN[0]
B8.VDDCR_SOC  B8.VDDCR_SOC  pwr
B9.DP2_TXP[3]  B9.DP2_TXP[3]
B10.DP2_TXN[3]  B10.DP2_TXN[3]
B11.VDDCR_SOC  B11.VDDCR_SOC  pwr
B12.TEST15  B12.TEST15
B13.TRST_L  B13.TRST_L
B14.VDDCR_SOC  B14.VDDCR_SOC  pwr
B15.TMS  B15.TMS
B16.RESET_L  B16.RESET_L
B17.VDDCR_SOC  B17.VDDCR_SOC  pwr
B18.SIC  B18.SIC
B19.VSS  B19.VSS  out
B20.VDDCR_SOC  B20.VDDCR_SOC  pwr
B21.MB_DATA[1]  B21.MB_DATA[1]
B22.MB_DQS_H[0]  B22.MB_DQS_H[0]
B23.VSS  B23.VSS  out
B24.MB_DATA[2]  B24.MB_DATA[2]
B25.MB_DATA[13]  B25.MB_DATA[13]
B26.VSS  B26.VSS  out
B27.MB_DQS_L[1]  B27.MB_DQS_L[1]
B28.MB_DATA[15]  B28.MB_DATA[15]
B29.VSS  B29.VSS  out
B30.MB_DATA[20]  B30.MB_DATA[20]
B31.MB_DATA[17]  B31.MB_DATA[17]
B32.VSS  B32.VSS  out
B33.MB_DATA[22]  B33.MB_DATA[22]
B34.MB_DATA[18]  B34.MB_DATA[18]
B35.VSS  B35.VSS  out
B36.MB_DATA[24]  B36.MB_DATA[24]
B37.MB_DQS_H[3]  B37.MB_DQS_H[3]
B38.MB_DATA[30]  B38.MB_DATA[30]
C1.VSS  C1.VSS  out
C2.DP0_TXN[0]  C2.DP0_TXN[0]
C3.DP0_TXP[1]  C3.DP0_TXP[1]
C4.VDDCR_SOC  C4.VDDCR_SOC  pwr
C5.DP0_TXP[3]  C5.DP0_TXP[3]
C6.DP0_TXN[3]  C6.DP0_TXN[3]
C7.VDDCR_SOC  C7.VDDCR_SOC  pwr
C8.DP2_TXP[2]  C8.DP2_TXP[2]
C9.DP2_TXN[2]  C9.DP2_TXN[2]
C10.VDDCR_SOC  C10.VDDCR_SOC  pwr
C11.TEST16  C11.TEST16
C12.TEST14  C12.TEST14
C13.VDDCR_SOC  C13.VDDCR_SOC  pwr
C14.TDO  C14.TDO
C15.TCK  C15.TCK
C16.VDDCR_SOC  C16.VDDCR_SOC  pwr
C17.SVD  C17.SVD
C18.SID  C18.SID
C19.VDDCR_SOC  C19.VDDCR_SOC  pwr
C20.MB_DATA[5]  C20.MB_DATA[5]
C21.MB_DM[0]  C21.MB_DM[0]
C22.VSS  C22.VSS  out
C23.MB_DATA[7]  C23.MB_DATA[7]
C24.MB_DATA[3]  C24.MB_DATA[3]
C25.VSS  C25.VSS  out
C26.MB_DATA[9]  C26.MB_DATA[9]
C27.MB_DQS_H[1]  C27.MB_DQS_H[1]
C28.VSS  C28.VSS  out
C29.MB_DATA[11]  C29.MB_DATA[11]
C30.MB_DATA[21]  C30.MB_DATA[21]
C31.VSS  C31.VSS  out
C32.MB_DQS_L[2]  C32.MB_DQS_L[2]
C33.MB_DQS_H[2]  C33.MB_DQS_H[2]
C34.VSS  C34.VSS  out
C35.MB_DATA[19]  C35.MB_DATA[19]
C36.MB_DATA[29]  C36.MB_DATA[29]
C37.VSS  C37.VSS  out
C38.MB_DATA[31]  C38.MB_DATA[31]
C39.MB_DATA[26]  C39.MB_DATA[26]
D1.P_GFX_TXP[0]  D1.P_GFX_TXP[0]
D2.DP0_TXP[0]  D2.DP0_TXP[0]
D3.VDDCR_SOC  D3.VDDCR_SOC  pwr
D4.DP1_TXP[0]  D4.DP1_TXP[0]
D5.DP1_TXN[0]  D5.DP1_TXN[0]
D6.VSS  D6.VSS  out
D7.DP1_TXP[1]  D7.DP1_TXP[1]
D8.DP1_TXN[1]  D8.DP1_TXN[1]
D9.VSS  D9.VSS  out
D10.DP1_HPD  D10.DP1_HPD
D11.TEST17  D11.TEST17
D12.VSS  D12.VSS  out
D13.TEST6  D13.TEST6
D14.DBREQ_L  D14.DBREQ_L
D15.VSS  D15.VSS  out
D16.ALERT_L  D16.ALERT_L
D17.SVC  D17.SVC
D18.VSS  D18.VSS  out
D19.VSS  D19.VSS  out
D20.MB_DATA[0]  D20.MB_DATA[0]
D21.VSS  D21.VSS  out
D22.VSS  D22.VSS  out
D23.VSS  D23.VSS  out
D24.VSS  D24.VSS  out
D25.VSS  D25.VSS  out
D26.MB_DM[1]  D26.MB_DM[1]
D27.VSS  D27.VSS  out
D28.RSVD  D28.RSVD  nc
D29.VSS  D29.VSS  out
D30.VSS  D30.VSS  out
D31.VSS  D31.VSS  out
D32.VSS  D32.VSS  out
D33.VSS  D33.VSS  out
D34.VSS  D34.VSS  out
D35.VSS  D35.VSS  out
D36.VSS  D36.VSS  out
D37.MB_DM[3]  D37.MB_DM[3]
D38.MB_DATA[27]  D38.MB_DATA[27]
D39.VSS  D39.VSS  out
E1.P_GFX_TXN[0]  E1.P_GFX_TXN[0]
E2.VDDCR_SOC  E2.VDDCR_SOC  pwr
E3.P_GFX_TXP[1]  E3.P_GFX_TXP[1]
E4.VSS  E4.VSS  out
E5.VSS  E5.VSS  out
E6.TEST28_H  E6.TEST28_H
E7.TEST28_L  E7.TEST28_L
E8.VSS  E8.VSS  out
E9.DP1_TXP[3]  E9.DP1_TXP[3]
E10.DP2_HPD  E10.DP2_HPD
E11.VSS  E11.VSS  out
E12.DP_AUX_ZVSS  E12.DP_AUX_ZVSS  out
E13.DBRDY  E13.DBRDY
E14.VSS  E14.VSS  out
E15.VDDCR_SOC_SENSE  E15.VDDCR_SOC_SENSE  pwr
E16.PWROK  E16.PWROK
E17.VSS  E17.VSS  out
E18.MA_DATA[0]  E18.MA_DATA[0]
E19.RSVD  E19.RSVD  nc
E20.VSS  E20.VSS  out
E21.VSS  E21.VSS  out
E22.RSVD  E22.RSVD  nc
E23.VSS  E23.VSS  out
E24.MA_DATA[10]  E24.MA_DATA[10]
E25.RSVD  E25.RSVD  nc
E26.VSS  E26.VSS  out
E27.VSS  E27.VSS  out
E28.MA_DATA[22]  E28.MA_DATA[22]
E29.VSS  E29.VSS  out
E30.MA_DQS_L[3]  E30.MA_DQS_L[3]
E31.MA_DATA[30]  E31.MA_DATA[30]
E32.VSS  E32.VSS  out
E33.MA_CHECK[4]  E33.MA_CHECK[4]
E34.MA_CHECK[5]  E34.MA_CHECK[5]
E35.VSS  E35.VSS  out
E36.MB_DATA[25]  E36.MB_DATA[25]
E37.MB_CHECK[4]  E37.MB_CHECK[4]
E38.VSS  E38.VSS  out
E39.MB_CHECK[5]  E39.MB_CHECK[5]
F1.VSS  F1.VSS  out
F2.P_GFX_TXP[2]  F2.P_GFX_TXP[2]
F3.P_GFX_TXN[1]  F3.P_GFX_TXN[1]
F4.VSS  F4.VSS  out
F5.P_GFX_RXN[0]  F5.P_GFX_RXN[0]
F6.P_GFX_RXP[0]  F6.P_GFX_RXP[0]
F7.VDDCR_SOC  F7.VDDCR_SOC  pwr
F8.DP1_TXP[2]  F8.DP1_TXP[2]
F9.DP1_TXN[3]  F9.DP1_TXN[3]
F10.VDDCR_SOC  F10.VDDCR_SOC  pwr
F11.DP1_AUXP  F11.DP1_AUXP
F12.DP_ZVSS  F12.DP_ZVSS  out
F13.VDDCR_SOC  F13.VDDCR_SOC  pwr
F14.VDDCR_CPU_SENSE  F14.VDDCR_CPU_SENSE  pwr
F15.VSS_SENSE_A  F15.VSS_SENSE_A
F16.VDDCR_SOC  F16.VDDCR_SOC  pwr
F17.VSS  F17.VSS  out
F18.MA_DATA[5]  F18.MA_DATA[5]
F19.VSS  F19.VSS  out
F20.MA_DATA[7]  F20.MA_DATA[7]
F21.MA_DATA[12]  F21.MA_DATA[12]
F22.VSS  F22.VSS  out
F23.MA_DQS_H[1]  F23.MA_DQS_H[1]
F24.MA_DATA[15]  F24.MA_DATA[15]
F25.VSS  F25.VSS  out
F26.MA_DQS_L[2]  F26.MA_DQS_L[2]
F27.MA_DQS_H[2]  F27.MA_DQS_H[2]
F28.VSS  F28.VSS  out
F29.MA_DATA[24]  F29.MA_DATA[24]
F30.MA_DQS_H[3]  F30.MA_DQS_H[3]
F31.VSS  F31.VSS  out
F32.MA_DATA[27]  F32.MA_DATA[27]
F33.MA_CHECK[0]  F33.MA_CHECK[0]
F34.VSS  F34.VSS  out
F35.VSS  F35.VSS  out
F36.MB_CHECK[1]  F36.MB_CHECK[1]
F37.VSS  F37.VSS  out
F38.MB_CHECK[0]  F38.MB_CHECK[0]
F39.MB_DM[8]  F39.MB_DM[8]
G1.P_GFX_TXP[3]  G1.P_GFX_TXP[3]
G2.P_GFX_TXN[2]  G2.P_GFX_TXN[2]
G3.VDDCR_SOC  G3.VDDCR_SOC  pwr
G4.P_GFX_RXN[1]  G4.P_GFX_RXN[1]
G5.P_GFX_RXP[1]  G5.P_GFX_RXP[1]
G6.VDDCR_SOC  G6.VDDCR_SOC  pwr
G7.VSS  G7.VSS  out
G8.DP1_TXN[2]  G8.DP1_TXN[2]
G9.VDDCR_SOC  G9.VDDCR_SOC  pwr
G10.DP0_AUXP  G10.DP0_AUXP
G11.DP1_AUXN  G11.DP1_AUXN
G12.VDDCR_SOC  G12.VDDCR_SOC  pwr
G13.DP_BLON  G13.DP_BLON
G14.VDDIO_MEM_S3_SENSE  G14.VDDIO_MEM_S3_SENSE  pwr
G15.VDDCR_SOC  G15.VDDCR_SOC  pwr
G16.TEST18  G16.TEST18
G17.RSVD  G17.RSVD  nc
G18.VDDCR_SOC  G18.VDDCR_SOC  pwr
G19.MA_DQS_L[0]  G19.MA_DQS_L[0]
G20.MA_DATA[6]  G20.MA_DATA[6]
G21.VSS  G21.VSS  out
G22.MA_DATA[9]  G22.MA_DATA[9]
G23.MA_DQS_L[1]  G23.MA_DQS_L[1]
G24.VSS  G24.VSS  out
G25.MA_DATA[21]  G25.MA_DATA[21]
G26.MA_DM[2]  G26.MA_DM[2]
G27.VSS  G27.VSS  out
G28.MA_DATA[18]  G28.MA_DATA[18]
G29.MA_DATA[29]  G29.MA_DATA[29]
G30.VSS  G30.VSS  out
G31.MA_DATA[31]  G31.MA_DATA[31]
G32.MA_CHECK[1]  G32.MA_CHECK[1]
G33.VSS  G33.VSS  out
G34.MA_DM[8]  G34.MA_DM[8]
G35.VSS  G35.VSS  out
G36.VSS  G36.VSS  out
G37.MB_DQS_L[8]  G37.MB_DQS_L[8]
G38.MB_DQS_H[8]  G38.MB_DQS_H[8]
G39.VSS  G39.VSS  out
H1.P_GFX_TXN[3]  H1.P_GFX_TXN[3]
H2.VDDCR_SOC  H2.VDDCR_SOC  pwr
H3.P_GFX_TXP[4]  H3.P_GFX_TXP[4]
H4.VSS  H4.VSS  out
H5.VSS  H5.VSS  out
H6.P_GFX_RXN[2]  H6.P_GFX_RXN[2]
H7.P_GFX_RXP[2]  H7.P_GFX_RXP[2]
H8.VSS  H8.VSS  out
H9.DP0_HPD  H9.DP0_HPD
H10.DP0_AUXN  H10.DP0_AUXN
H11.VSS  H11.VSS  out
H12.DP_VARYBL  H12.DP_VARYBL
H13.DP_DIGON  H13.DP_DIGON
H14.VSS  H14.VSS  out
H15.PROCHOT_L  H15.PROCHOT_L
H16.TEST19  H16.TEST19
H17.VSS  H17.VSS  out
H18.MA_DATA[4]  H18.MA_DATA[4]
H19.MA_DQS_H[0]  H19.MA_DQS_H[0]
H20.VSS  H20.VSS  out
H21.MA_DATA[3]  H21.MA_DATA[3]
H22.MA_DATA[8]  H22.MA_DATA[8]
H23.VSS  H23.VSS  out
H24.MA_DATA[14]  H24.MA_DATA[14]
H25.MA_DATA[20]  H25.MA_DATA[20]
H26.VSS  H26.VSS  out
H27.MA_DATA[23]  H27.MA_DATA[23]
H28.MA_DATA[19]  H28.MA_DATA[19]
H29.VSS  H29.VSS  out
H30.MA_DM[3]  H30.MA_DM[3]
H31.MA_DATA[26]  H31.MA_DATA[26]
H32.VSS  H32.VSS  out
H33.MA_DQS_L[8]  H33.MA_DQS_L[8]
H34.MA_DQS_H[8]  H34.MA_DQS_H[8]
H35.VSS  H35.VSS  out
H36.MB_CHECK[6]  H36.MB_CHECK[6]
H37.MB_CHECK[7]  H37.MB_CHECK[7]
H38.VSS  H38.VSS  out
H39.MB_CHECK[2]  H39.MB_CHECK[2]
J1.VSS  J1.VSS  out
J2.P-GFX_TXP[5]  J2.P-GFX_TXP[5]
J3.P_GFX_TXN[4]  J3.P_GFX_TXN[4]
J4.VSS  J4.VSS  out
J5.P_GFX_RXN[3]  J5.P_GFX_RXN[3]
J6.P_GFX_RXP[3]  J6.P_GFX_RXP[3]
J7.VDDCR_SOC  J7.VDDCR_SOC  pwr
J8.VSS  J8.VSS  out
J9.VSS  J9.VSS  out
J10.VDDCR_SOC  J10.VDDCR_SOC  pwr
J11.VSS  J11.VSS  out
J12.VDDCR_SOC  J12.VDDCR_SOC  pwr
J13.VSS  J13.VSS  out
J14.VDDCR_SOC  J14.VDDCR_SOC  pwr
J15.VSS  J15.VSS  out
J16.VDDCR_SOC  J16.VDDCR_SOC  pwr
J17.VSS  J17.VSS  out
J18.MA_DATA[1]  J18.MA_DATA[1]
J19.VSS  J19.VSS  out
J20.MA_DATA[2]  J20.MA_DATA[2]
J21.MA_DATA[13]  J21.MA_DATA[13]
J22.VSS  J22.VSS  out
J23.MA_DM[1]  J23.MA_DM[1]
J24.MA_DATA[11]  J24.MA_DATA[11]
J25.VSS  J25.VSS  out
J26.MA_DATA[16]  J26.MA_DATA[16]
J27.MA_DATA[17]  J27.MA_DATA[17]
J28.VSS  J28.VSS  out
J29.MA_DATA[28]  J29.MA_DATA[28]
J30.MA_DATA[25]  J30.MA_DATA[25]
J31.VSS  J31.VSS  out
J32.MA_CHECK[6]  J32.MA_CHECK[6]
J33.MA_CHECK[7]  J33.MA_CHECK[7]
J34.VSS  J34.VSS  out
J35.VSS  J35.VSS  out
J36.RSVD  J36.RSVD  nc
J37.VSS  J37.VSS  out
J38.RSVD  J38.RSVD  nc
J39.MB_CHECK[3]  J39.MB_CHECK[3]
K1.P_GFX_TXP[6]  K1.P_GFX_TXP[6]
K2.P_GFX_TXN[5]  K2.P_GFX_TXN[5]
K3.VDDCR_SOC  K3.VDDCR_SOC  pwr
K4.P_GFX_RXN[5]  K4.P_GFX_RXN[5]
K5.P_GFX_RXP[5]  K5.P_GFX_RXP[5]
K6.VDDCR_SOC  K6.VDDCR_SOC  pwr
K7.P_GFX_RXN[4]  K7.P_GFX_RXN[4]
K8.P_GFX_RXP[4]  K8.P_GFX_RXP[4]
K9.VDDCR_SOC  K9.VDDCR_SOC  pwr
K10.VSS  K10.VSS  out
K11.VDDCR_SOC  K11.VDDCR_SOC  pwr
K12.VSS  K12.VSS  out
K13.VDDCR_SOC  K13.VDDCR_SOC  pwr
K14.DP_STEREOSYNC  K14.DP_STEREOSYNC
K15.VDDCR_SOC  K15.VDDCR_SOC  pwr
K18.VSS  K18.VSS  out
K19.MA_DM[0]  K19.MA_DM[0]
K20.VSS  K20.VSS  out
K21.VSS  K21.VSS  out
K22.VSS  K22.VSS  out
K23.VSS  K23.VSS  out
K26.VSS  K26.VSS  out
K27.VSS  K27.VSS  out
K28.VSS  K28.VSS  out
K29.VSS  K29.VSS  out
K30.VSS  K30.VSS  out
K31.MA_CHECK[2]  K31.MA_CHECK[2]
K32.MA_CHECK[3]  K32.MA_CHECK[3]
K33.VSS  K33.VSS  out
K34.RSVD  K34.RSVD  nc
K35.MB_RESET_L  K35.MB_RESET_L
K36.VDDIO_MEM_S3  K36.VDDIO_MEM_S3  pwr
K37.MB0_CKE[1]  K37.MB0_CKE[1]
K38.RSVD  K38.RSVD  nc
K39.VDDIO_MEM_S3  K39.VDDIO_MEM_S3  pwr
L1.P_GFX_TXN[6]  L1.P_GFX_TXN[6]
L2.VDDCR_SOC  L2.VDDCR_SOC  pwr
L3.P_GFX_TXP[7]  L3.P_GFX_TXP[7]
L4.VSS  L4.VSS  out
L5.VSS  L5.VSS  out
L6.P_GFX_RXN[6]  L6.P_GFX_RXN[6]
L7.P_GFX_RXP[6]  L7.P_GFX_RXP[6]
L8.VSS  L8.VSS  out
L9.VSS  L9.VSS  out
L10.VDDCR_SOC  L10.VDDCR_SOC  pwr
L11.VSS  L11.VSS  out
L12.VDDCR_SOC  L12.VDDCR_SOC  pwr
L13.VSS  L13.VSS  out
L14.VDDCR_SOC  L14.VDDCR_SOC  pwr
L15.VSS  L15.VSS  out
L16.VDDCR_SOC  L16.VDDCR_SOC  pwr
L17.VSS  L17.VSS  out
L18.VDDCR_SOC  L18.VDDCR_SOC  pwr
L19.VSS  L19.VSS  out
L20.VDDCR_SOC  L20.VDDCR_SOC  pwr
L21.VSS  L21.VSS  out
L22.VDDCR_SOC  L22.VDDCR_SOC  pwr
L23.TEST4  L23.TEST4
L24.VDDCR_SOC  L24.VDDCR_SOC  pwr
L25.VSS  L25.VSS  out
L26.VDDCR_SOC  L26.VDDCR_SOC  pwr
L27.VSS  L27.VSS  out
L28.VSS  L28.VSS  out
L29.VSS  L29.VSS  out
L30.VSS  L30.VSS  out
L31.VSS  L31.VSS  out
L32.VDDIO_MEM_S3  L32.VDDIO_MEM_S3  pwr
L33.MA_RESET_L  L33.MA_RESET_L
L34.MA1_CKE[1]  L34.MA1_CKE[1]
L35.VDDIO_MEM_S3  L35.VDDIO_MEM_S3  pwr
L36.MB1_CKE[1]  L36.MB1_CKE[1]
L37.MB0_CKE[0]  L37.MB0_CKE[0]
L38.VDDIO_MEM_S3  L38.VDDIO_MEM_S3  pwr
L39.MB1_CKE[0]  L39.MB1_CKE[0]
M1.VSS  M1.VSS  out
M2.P_GFX_TXP[8]  M2.P_GFX_TXP[8]
M3.P_GFX_TXN[7]  M3.P_GFX_TXN[7]
M4.VSS  M4.VSS  out
M5.P_GFX_RXN[7]  M5.P_GFX_RXN[7]
M6.P_GFX_RXP[7]  M6.P_GFX_RXP[7]
M7.VDDCR_CPU  M7.VDDCR_CPU  pwr
M8.VSS  M8.VSS  out
M9.VDDCR_SOC  M9.VDDCR_SOC  pwr
M10.VSS  M10.VSS  out
M11.VDDCR_SOC  M11.VDDCR_SOC  pwr
M12.VSS  M12.VSS  out
M13.VDDCR_SOC  M13.VDDCR_SOC  pwr
M14.VSS  M14.VSS  out
M15.VDDCR_SOC  M15.VDDCR_SOC  pwr
M16.VSS  M16.VSS  out
M17.VDDCR_SOC  M17.VDDCR_SOC  pwr
M18.VSS  M18.VSS  out
M19.VDDCR_SOC  M19.VDDCR_SOC  pwr
M20.VSS  M20.VSS  out
M21.VDDCR_SOC  M21.VDDCR_SOC  pwr
M22.TEST5  M22.TEST5
M23.VDDCR_SOC  M23.VDDCR_SOC  pwr
M24.VSS  M24.VSS  out
M25.VDDCR_SOC  M25.VDDCR_SOC  pwr
M26.VSS  M26.VSS  out
M27.VSS  M27.VSS  out
M28.VSS  M28.VSS  out
M29.VDDIO_MEM_S3  M29.VDDIO_MEM_S3  pwr
M30.MA0_CKE[1]  M30.MA0_CKE[1]
M31.VDDIO_MEM_S3  M31.VDDIO_MEM_S3  pwr
M32.MA0_CKE[0]  M32.MA0_CKE[0]
M33.MA1_CKE[0]  M33.MA1_CKE[0]
M34.VDDIO_MEM_S3  M34.VDDIO_MEM_S3  pwr
M35.MA_ACT_L  M35.MA_ACT_L
M36.MB_BG[0]  M36.MB_BG[0]
M37.VDDIO_MEM_S3  M37.VDDIO_MEM_S3  pwr
M38.MB_ACT_L  M38.MB_ACT_L
M39.MB_BG[1]  M39.MB_BG[1]
N1.P_GFX_TXP[9]  N1.P_GFX_TXP[9]
N2.P_GFX_TXN[8]  N2.P_GFX_TXN[8]
N3.VDDCR_CPU  N3.VDDCR_CPU  pwr
N4.P_GFX_RXN[9]  N4.P_GFX_RXN[9]
N5.P_GFX_RXP[9]  N5.P_GFX_RXP[9]
N6.VDDCR_CPU  N6.VDDCR_CPU  pwr
N7.P_GFX_RXN[8]  N7.P_GFX_RXN[8]
N8.P_GFX_RXP[8]  N8.P_GFX_RXP[8]
N9.VSS  N9.VSS  out
N10.VDDCR_SOC  N10.VDDCR_SOC  pwr
N11.VSS  N11.VSS  out
N12.VDDCR_SOC  N12.VDDCR_SOC  pwr
N13.VSS  N13.VSS  out
N14.VDDCR_SOC  N14.VDDCR_SOC  pwr
N15.VSS  N15.VSS  out
N16.VDDCR_SOC  N16.VDDCR_SOC  pwr
N17.VSS  N17.VSS  out
N18.VDDCR_SOC  N18.VDDCR_SOC  pwr
N19.VSS  N19.VSS  out
N20.VDDCR_SOC  N20.VDDCR_SOC  pwr
N21.VSS  N21.VSS  out
N22.VDDCR_SOC  N22.VDDCR_SOC  pwr
N23.VSS  N23.VSS  out
N24.VDDCR_SOC  N24.VDDCR_SOC  pwr
N25.VSS  N25.VSS  out
N26.VDDCR_SOC  N26.VDDCR_SOC  pwr
N27.VSS  N27.VSS  out
N28.VDDIO_MEM_S3  N28.VDDIO_MEM_S3  pwr
N29.VSS  N29.VSS  out
N30.VDDIO_MEM_S3  N30.VDDIO_MEM_S3  pwr
N31.MA_BG[0]  N31.MA_BG[0]
N32.MA_BG[1]  N32.MA_BG[1]
N33.VDDIO_MEM_S3  N33.VDDIO_MEM_S3  pwr
N34.MA_ALERT_L  N34.MA_ALERT_L
N35.MA_ADD[12]  N35.MA_ADD[12]
N36.VDDIO_MEM_S3  N36.VDDIO_MEM_S3  pwr
N37.MB_ALERT_L  N37.MB_ALERT_L
N38.MB_ADD[12]  N38.MB_ADD[12]
N39.VDDIO_MEM_S3  N39.VDDIO_MEM_S3  pwr
P1.P_GFX_TXN[9]  P1.P_GFX_TXN[9]
P2.VDDCR_CPU  P2.VDDCR_CPU  pwr
P3.P_GFX_TXP[10]  P3.P_GFX_TXP[10]
P4.VSS  P4.VSS  out
P5.VSS  P5.VSS  out
P6.P_GFX_RXN[10]  P6.P_GFX_RXN[10]
P7.P_GFX_RXP[10]  P7.P_GFX_RXP[10]
P8.VSS  P8.VSS  out
P9.VDDCR_SOC  P9.VDDCR_SOC  pwr
P10.VSS  P10.VSS  out
P11.VDDCR_SOC  P11.VDDCR_SOC  pwr
P12.VSS  P12.VSS  out
P13.VDDCR_SOC  P13.VDDCR_SOC  pwr
P27.VDDIO_MEM_S3  P27.VDDIO_MEM_S3  pwr
P28.TEST47  P28.TEST47
P29.VDDIO_MEM_S3  P29.VDDIO_MEM_S3  pwr
P30.MA_ADD[8]  P30.MA_ADD[8]
P31.MA_ADD[9]  P31.MA_ADD[9]
P32.VDDIO_MEM_S3  P32.VDDIO_MEM_S3  pwr
P33.MA_ADD[11]  P33.MA_ADD[11]
P34.MA_ADD[7]  P34.MA_ADD[7]
P35.VDDIO_MEM_S3  P35.VDDIO_MEM_S3  pwr
P36.MB_ADD[9]  P36.MB_ADD[9]
P37.MB_ADD[11]  P37.MB_ADD[11]
P38.VDDIO_MEM_S3  P38.VDDIO_MEM_S3  pwr
P39.MB_ADD[7]  P39.MB_ADD[7]
R1.VSS  R1.VSS  out
R2.P_GFX_TXP[11]  R2.P_GFX_TXP[11]
R3.P_GFX_TXN[10]  R3.P_GFX_TXN[10]
R4.VSS  R4.VSS  out
R5.P_GFX_RXN[11]  R5.P_GFX_RXN[11]
R6.P_GFX_RXP[11]  R6.P_GFX_RXP[11]
R7.VDDCR_CPU  R7.VDDCR_CPU  pwr
R8.VSS  R8.VSS  out
R9.VSS  R9.VSS  out
R10.VDDCR-SOC  R10.VDDCR-SOC  pwr
R11.VSS  R11.VSS  out
R12.VDDCR_SOC  R12.VDDCR_SOC  pwr
R13.VSS  R13.VSS  out
R27.VSS  R27.VSS  out
R28.VDDIO_MEM_S3  R28.VDDIO_MEM_S3  pwr
R29.VSS  R29.VSS  out
R30.MA_ADD[4]  R30.MA_ADD[4]
R31.VDDIO_MEM_S3  R31.VDDIO_MEM_S3  pwr
R32.MA_ADD[6]  R32.MA_ADD[6]
R33.MA_ADD[5]  R33.MA_ADD[5]
R34.VDDIO_MEM_S3  R34.VDDIO_MEM_S3  pwr
R35.RSVD  R35.RSVD  nc
R36.MB_ADD[6]  R36.MB_ADD[6]
R37.VDDIO_MEM_S3  R37.VDDIO_MEM_S3  pwr
R38.MB_ADD[8]  R38.MB_ADD[8]
R39.MB_ADD[5]  R39.MB_ADD[5]
T1.P_GFX_TXP[12]  T1.P_GFX_TXP[12]
T2.P_GFX_TXN[11]  T2.P_GFX_TXN[11]
T3.VDDCR_CPU  T3.VDDCR_CPU  pwr
T4.P_GFX_RXP[13]  T4.P_GFX_RXP[13]
T5.P_GFX_RXN[13]  T5.P_GFX_RXN[13]
T6.VDDCR_CPU  T6.VDDCR_CPU  pwr
T7.P_GFX_RXN[12]  T7.P_GFX_RXN[12]
T8.P_GFX_RXP[12]  T8.P_GFX_RXP[12]
T9.VDDCR_CPU  T9.VDDCR_CPU  pwr
T10.VSS  T10.VSS  out
T11.VDDCR_SOC  T11.VDDCR_SOC  pwr
T12.VSS  T12.VSS  out
T13.VDDCR_SOC  T13.VDDCR_SOC  pwr
T27.VDDIO_MEM_S3  T27.VDDIO_MEM_S3  pwr
T28.VSS  T28.VSS  out
T29.VDDIO_MEM_S3  T29.VDDIO_MEM_S3  pwr
T30.VSS  T30.VSS  out
T31.MA_ADD[3]  T31.MA_ADD[3]
T32.MA_ADD[1]  T32.MA_ADD[1]
T33.VDDIO_MEM_S3  T33.VDDIO_MEM_S3  pwr
T34.MA_CLK_H[0]  T34.MA_CLK_H[0]
T35.MA_ADD[2]  T35.MA_ADD[2]
T36.VDDIO_MEM_S3  T36.VDDIO_MEM_S3  pwr
T37.MB_ADD[4]  T37.MB_ADD[4]
T38.MB_ADD[3]  T38.MB_ADD[3]
T39.VDDIO_MEM_S3  T39.VDDIO_MEM_S3  pwr
U1.P_GFX_TXN[12]  U1.P_GFX_TXN[12]
U2.VDDCR_CPU  U2.VDDCR_CPU  pwr
U3.P_GFX_TXP[13]  U3.P_GFX_TXP[13]
U4.VSS  U4.VSS  out
U5.VSS  U5.VSS  out
U6.P_GFX_RXN[14]  U6.P_GFX_RXN[14]
U7.P_GFX_RXP[14]  U7.P_GFX_RXP[14]
U8.VSS  U8.VSS  out
U9.VSS  U9.VSS  out
U10.VDDCR_CPU  U10.VDDCR_CPU  pwr
U11.VSS  U11.VSS  out
U12.VDDCR_SOC  U12.VDDCR_SOC  pwr
U13.VSS  U13.VSS  out
U27.VSS  U27.VSS  out
U28.VDDIO_MEM_S3  U28.VDDIO_MEM_S3  pwr
U29.VSS  U29.VSS  out
U30.VDDIO_MEM_S3  U30.VDDIO_MEM_S3  pwr
U31.VSS  U31.VSS  out
U32.VDDIO_MEM_S3  U32.VDDIO_MEM_S3  pwr
U33.MA_CLK_H[1]  U33.MA_CLK_H[1]
U34.MA_CLK_L[0]  U34.MA_CLK_L[0]
U35.VDDIO_MEM_S3  U35.VDDIO_MEM_S3  pwr
U36.MB_ADD[1]  U36.MB_ADD[1]
U37.MB_ADD[2]  U37.MB_ADD[2]
U38.VDDIO_MEM_S3  U38.VDDIO_MEM_S3  pwr
U39.MB_CLK_H[0]  U39.MB_CLK_H[0]
V1.VSS  V1.VSS  out
V2.P_GFX_TXP[14]  V2.P_GFX_TXP[14]
V3.P_GFX_TXN[13]  V3.P_GFX_TXN[13]
V4.VSS  V4.VSS  out
V5.P_GFX_RXN[15]  V5.P_GFX_RXN[15]
V6.P_GFX_RXP[15]  V6.P_GFX_RXP[15]
V7.VSS  V7.VSS  out
V8.P0A_ZVSS  V8.P0A_ZVSS  out
V9.VDDCR_CPU  V9.VDDCR_CPU  pwr
V10.VSS  V10.VSS  out
V11.VDDCR_CPU  V11.VDDCR_CPU  pwr
V12.VSS  V12.VSS  out
V13.VDDCR_SOC  V13.VDDCR_SOC  pwr
V27.VDDIO_MEM_S3  V27.VDDIO_MEM_S3  pwr
V28.VSS  V28.VSS  out
V29.VDDIO_MEM_S3  V29.VDDIO_MEM_S3  pwr
V30.VSS  V30.VSS  out
V31.VDDIO_MEM_S3  V31.VDDIO_MEM_S3  pwr
V32.MA_CLK_H[3]  V32.MA_CLK_H[3]
V33.MA_CLK_L[1]  V33.MA_CLK_L[1]
V34.VDDIO_MEM_S3  V34.VDDIO_MEM_S3  pwr
V35.MA_CLK_H[2]  V35.MA_CLK_H[2]
V36.MA_CLK_L[2]  V36.MA_CLK_L[2]
V37.VDDIO_MEM_S3  V37.VDDIO_MEM_S3  pwr
V38.MB_CLK_H[1]  V38.MB_CLK_H[1]
V39.MB_CLK_L[0]  V39.MB_CLK_L[0]
W1.P_GFX_TXP[15]  W1.P_GFX_TXP[15]
W2.P_GFX_TXN[14]  W2.P_GFX_TXN[14]
W3.VDDCR_CPU  W3.VDDCR_CPU  pwr
W4.P_HUB_RXP[3]  W4.P_HUB_RXP[3]
W5.P_HUB_RXN[3]  W5.P_HUB_RXN[3]
W6.VDDCR_CPU  W6.VDDCR_CPU  pwr
W7.P_ZVSS  W7.P_ZVSS  out
W8.P_ZVDDP  W8.P_ZVDDP  pwr
W9.VSS  W9.VSS  out
W10.VDDCR_CPU  W10.VDDCR_CPU  pwr
W11.VSS  W11.VSS  out
W12.VDDCR_CPU  W12.VDDCR_CPU  pwr
W13.VSS  W13.VSS  out
W27.VSS  W27.VSS  out
W28.VDDIO_MEM_S3  W28.VDDIO_MEM_S3  pwr
W29.VSS  W29.VSS  out
W30.TEST40  W30.TEST40
W31.VSS  W31.VSS  out
W32.MA_CLK_L[3]  W32.MA_CLK_L[3]
W33.VDDIO_MEM_S3  W33.VDDIO_MEM_S3  pwr
W34.VDDIO_MEM_S3  W34.VDDIO_MEM_S3  pwr
W35.MA_EVENT_L  W35.MA_EVENT_L
W36.VDDIO_MEM_S3  W36.VDDIO_MEM_S3  pwr
W37.MB_CLK_H[2]  W37.MB_CLK_H[2]
W38.MB_CLK_L[1]  W38.MB_CLK_L[1]
W39.VDDIO_MEM_S3  W39.VDDIO_MEM_S3  pwr
Y1.P_GFX_TXN[15]  Y1.P_GFX_TXN[15]
Y2.VDDCR_CPU  Y2.VDDCR_CPU  pwr
Y3.USB_SS_0RXP  Y3.USB_SS_0RXP
Y4.USB_SS_0RXN  Y4.USB_SS_0RXN
Y5.VSS  Y5.VSS  out
Y6.P_HUB_RXP[2]  Y6.P_HUB_RXP[2]
Y7.P_HUB_RXN[2]  Y7.P_HUB_RXN[2]
Y8.VSS  Y8.VSS  out
Y9.VDDCR_CPU  Y9.VDDCR_CPU  pwr
Y10.VSS  Y10.VSS  out
Y11.VDDCR_CPU  Y11.VDDCR_CPU  pwr
Y12.VSS  Y12.VSS  out
Y13.VDDCR_CPU  Y13.VDDCR_CPU  pwr
Y27.VDDIO_MEM_S3  Y27.VDDIO_MEM_S3  pwr
Y28.VSS  Y28.VSS  out
Y29.VDDIO_MEM_S3  Y29.VDDIO_MEM_S3  pwr
Y30.VSS  Y30.VSS  out
Y31.VDDIO_MEM_S3  Y31.VDDIO_MEM_S3  pwr
Y32.VDDIO_MEM_S3  Y32.VDDIO_MEM_S3  pwr
Y33.MA_PARTOUT  Y33.MA_PARTOUT  out
Y34.MA__ZVDDIO_MEM_S3  Y34.MA__ZVDDIO_MEM_S3  pwr
Y35.VDDIO_MEM_S3  Y35.VDDIO_MEM_S3  pwr
Y36.MB__ZVDDIO_MEM_S3  Y36.MB__ZVDDIO_MEM_S3  pwr
Y37.MB_CLK_L[2]  Y37.MB_CLK_L[2]
Y38.VDDIO_MEM_S3  Y38.VDDIO_MEM_S3  pwr
Y39.MB_CLK_H[3]  Y39.MB_CLK_H[3]

## Footprint AM4_SOCKET (pad centres in mm)
Here is le pièce de résistance, AMD's 1331 pin AM4 Socket in all its glory. I named every pin by hand :P Shaped and Based on the Foxconn PZ1331A-51ZZ0-1H AM4 Socket by the one and only, YeaTheMen
smd 0.485 x 0.485: A3.VSS -17,19; AG1.VSS -19,-7; AH1.X48M_X2 -19,-8; AJ1.X48M_X1 -19,-9; AL1.USB_OC0_L/AGPIO16 -19,-11; AM1.USB_OC1_L/TDI/AGPIO17 -19,-12; AN1.VSS -19,-13; AP1.USB_OC3_L/TDO/AGPIO24 -19,-14; AR1.USB_OC2_L/TCK/AGPIO18 -19,-15; AT1.VSS -19,-16; AU1.AZ_RST_L -19,-17; AV2.VSS -18,-18; AW3.AZ_BITCLK -17,-19; B3.DP0_TXN[1] -17,18; C1.VSS -19,17; D1.P_GFX_TXP[0] -19,16; E1.P_GFX_TXN[0] -19,15; F1.VSS -19,14; G1.P_GFX_TXP[3] -19,13; H1.P_GFX_TXN[3] -19,12; J1.VSS -19,11; L1.P_GFX_TXN[6] -19,9; M1.VSS -19,8; N1.P_GFX_TXP[9] -19,7
smd 0.485 x 0.458: A4.DP0_TXN[2] -16,19; A5.RSVD -15,19; A6.VSS -14,19; A7.DP2_TXP[1] -13,19; A8.DP2_TXN[1] -12,19; A9.VSS -11,19; A10.DP2_AUXP -10,19; A11.DP2_AUXN -9,19; A12.VSS -8,19; A13.TEST11 -7,19; A14.TDI -6,19; A15.VSS -5,19; A16.TEST41 -4,19; A17.SVT -3,19; A18.VSS -2,19; A19.THERMTRIP_L -1,19; A20.MB_DATA[4] 0,19; A21.VSS 1,19; A22.MB_DQS_L[0] 2,19; A23.MB_DATA[6] 3,19; A24.VSS 4,19; A25.MB_DATA[12] 5,19; A26.MB_DATA[8] 6,19; A27.VSS 7,19; A28.MB_DATA[14] 8,19; A29.MB_DATA[10] 9,19; A30.VSS 10,19; A31.MB_DATA[16] 11,19; A32.MB_DM[2] 12,19; A33.VSS 13,19; A34.MB_DATA[23] 14,19; A35.MB_DATA[28] 15,19; A36.VSS 16,19; A37.MB_DQS_L[3] 17,19; AA1.VSS -19,-1; AA2.USB_SS_1RXP -18,-1; AA3.USB_SS_1RXN -17,-1; AA4.VSS -16,-1; AA5.P_HUB_TXP[1] -15,-1; AA6.VSS -14,-1; AA7.VDDCR_CPU -13,-1; AA8.P_HUB_RXN[1] -12,-1; AA9.VSS -11,-1; AA10.VDDCR_CPU -10,-1; AA11.VSS -9,-1; AA12.VDDCR_CPU -8,-1; AA13.VSS -7,-1; AA27.VSS 7,-1; AA28.VDDIO_MEM_S3 8,-1; AA29.VSS 9,-1; AA30.TEST31 10,-1; AA31.VSS 11,-1; AA32.MA_ADD[0] 12,-1; AA33.MA_BANK[1] 13,-1; AA34.VDDIO_MEM_S3 14,-1; AA35.MA_BANK[0] 15,-1; AA36.MA_ADD[10] 16,-1; AA37.VDDIO_MEM_S3 17,-1; AA38.MB_EVENT_L 18,-1; AA39.MB_CLK_L[3] 19,-1; AB1.USB_SS_1TXP -19,-2; AB2.RSVD -18,-2; AB3.VDDCR_CPU -17,-2; AB4.TEST10 -16,-2; AB5.P_HUB_TXN[1] -15,-2; AB6.VDDCR_CPU -14,-2; AB7.VSS -13,-2; AB8.P_HUB_RXP[1] -12,-2; AB9.VDDCR_CPU -11,-2; AB10.VSS -10,-2; AB11.VDDCR_CPU -9,-2; AB12.VSS -8,-2; AB13.VDDCR_CPU -7,-2; AB27.VDDIO_MEM_S3 7,-2; AB28.VSS 8,-2; AB29.VDDIO_MEM_S3 9,-2; AB30.VSS 10,-2; AB31.VDDIO_MEM_S3 11,-2; AB32.VDDIO_MEM_S3 12,-2; AB33.VDDIO_MEM_S3 13,-2; AB34.MA_RAS_L_ADD[16] 14,-2; AB35.MA_WE_L_ADD[14] 15,-2; AB36.VDDIO_MEM_S3 16,-2; AB37.RSVD 17,-2; AB38.MB_PARTOUT 18,-2; AB39.VDDIO_MEM_S3 19,-2; AC1.USB_SS_1TXN -19,-3; AC2.VDDCR_CPU -18,-3; AC3.USB_SS_2TXP -17,-3; AC4.USB_SS_2TXN -16,-3; AC5.VSS -15,-3; AC6.P_HUB_TXP[2] -14,-3; AC7.P_HUB_TXN[2] -13,-3; AC8.VSS -12,-3; AC9.VSS -11,-3; AC10.VDDCR_CPU -10,-3; AC11.VSS -9,-3; AC12.VDDCR_CPU -8,-3; AC13.VSS -7,-3; AC27.VSS 7,-3; AC28.VDDIO_MEM_S3 8,-3; AC29.VSS 9,-3; AC30.VDDIO_MEM_S3 10,-3; AC31.VSS 11,-3; AC32.VDDIO_MEM_S3 12,-3; AC33.MA0_CS_L[0] 13,-3; AC34.MA1_CS_L[0] 14,-3; AC35.VDDIO_MEM_S3 15,-3; AC36.MB_ADD[0] 16,-3; AC37.MB_BANK[1] 17,-3; AC38.VDDIO_MEM_S3 18,-3; AC39.MB_ADD[10] 19,-3; AD1.VSS -19,-4; AD2.USB_SS_3RXP -18,-4; AD3.RSVD -17,-4; AD4.VSS -16,-4; AD5.P_HUB_TXP[3] -15,-4; AD6.P_HUB_TXN[3] -14,-4; AD7.VDDCR_CPU -13,-4; AD8.P_HUB_RXN[0] -12,-4; AD9.VDDCR_CPU -11,-4; AD10.VSS -10,-4; AD11.VDDCR_CPU -9,-4; AD12.VSS -8,-4; AD13.VDDCR_CPU -7,-4; AD27.VDDIO_MEM_S3 7,-4; AD28.VSS 8,-4; AD29.VDDIO_MEM_S3 9,-4; AD30.VSS 10,-4; AD31.VDDIO_MEM_S3 11,-4; AD32.MA_CAS_L_ADD[15] 12,-4; AD33.MA1_ODT[0] 13,-4; AD34.VDDIO_MEM_S3 14,-4; AD35.MA0_ODT[0] 15,-4; AD36.MB_RAS_L_ADD[16] 16,-4; AD37.VDDIO_MEM_S3 17,-4; AD38.MB_BANK[0] 18,-4; AD39.MB_WE_L_ADD[14] 19,-4; AE1.USB_SS_3RXP -19,-5; AE2.USB_SS_2RXN -18,-5; AE3.VDDCR_CPU -17,-5; AE4.P_HUB_TXP[0] -16,-5; AE5.P_HUB_TXN[0] -15,-5; AE6.VDDCR_CPU -14,-5; AE7.VSS -13,-5; AE8.P_HUB_RXP[0] -12,-5; AE9.VSS -11,-5; AE10.VDDCR_CPU -10,-5; AE11.VSS -9,-5; AE12.VDDCR_CPU -8,-5; AE13.VSS -7,-5; AE27.VSS 7,-5; AE28.VDDIO_MEM_S3 8,-5; AE29.VSS 9,-5; AE30.VDDIO_MEM_S3 10,-5; AE31.VSS 11,-5; AE32.MA_ADD[13] 12,-5; AE33.VDDIO_MEM_S3 13,-5; AE34.MA1_CS_L[1] 14,-5; AE35.MA0_CS_L[1] 15,-5; AE36.VDDIO_MEM_S3 16,-5; AE37.MB0_CS_L[0] 17,-5; AE38.MB1_CS_L[0] 18,-5; AE39.VDDIO_MEM_S3 19,-5; AF1.USB_SS_3RXN -19,-6; AF2.VDDCR_CPU -18,-6; AF3.USB_SS_0TXP -17,-6; AF4.USB_SS_0TXN -16,-6; AF5.VSS -15,-6; AF6.GFX_CLKP -14,-6; AF7.GFX_CLKN -13,-6; AF8.VSS -12,-6; AF9.VDDCR_CPU -11,-6; AF10.VSS -10,-6; AF11.VDDCR_CPU -9,-6; AF12.VSS -8,-6; AF13.VDDCR_CPU -7,-6; AF27.VDDIO_MEM_S3 7,-6; AF28.VSS 8,-6; AF29.VDDIO_MEM_S3 9,-6; AF30.VSS 10,-6; AF31.MA0_ODT[1] 11,-6; AF32.VDDIO_MEM_S3 12,-6; AF33.MA_ADD_17 13,-6; AF34.MA1_ODT[1] 14,-6; AF35.VDDIO_MEM_S3 15,-6; AF36.MB_CAS_L_ADD[15] 16,-6; AF37.MB1_ODT[0] 17,-6; AF38.VDDIO_MEM_S3 18,-6; AF39.MB0_ODT[0] 19,-6; AG2.USB_SS_3TXP -18,-7; AG3.USB_SS_3TXN -17,-7; AG4.VSS -16,-7; AG5.GPP_CLK0P -15,-7; AG6.GPP_CLK0N -14,-7; AG7.VDDCR_CPU -13,-7; AG8.VSS -12,-7; AG9.VSS -11,-7; AG10.VDDCR_CPU -10,-7; AG11.VSS -9,-7; AG12.VDDCR_CPU -8,-7; AG13.VSS -7,-7; AG14.VDDCR_CPU -6,-7; AG15.VSS -5,-7; AG16.VDDCR_CPU -4,-7; AG17.VSS -3,-7; AG18.VDDCR_CPU -2,-7; AG19.VSS -1,-7; AG20.VDDCR_CPU 0,-7; AG21.VSS 1,-7; AG22.VDDCR_CPU 2,-7; AG23.VSS 3,-7; AG24.VDDCR_CPU 4,-7; AG25.VSS 5,-7; AG26.VDDCR_CPU 6,-7; AG27.VSS 7,-7; AG28.VSS 8,-7; AG29.VSS 9,-7; AG30.VSS 10,-7; AG31.VSS 11,-7; AG32.VSS 12,-7; AG33.VDDIO_MEM_S3 13,-7; AG34.VDDIO_MEM_S3 14,-7; AG35.VDDIO_MEM_S3 15,-7; AG36.MB1_CS_L[1] 16,-7; AG37.VDDIO_MEM_S3 17,-7; AG38.MB_ADD[13] 18,-7; AG39.MB0_CS_L[1] 19,-7; AH2.RSVD -18,-8; AH3.VDDCR_CPU -17,-8; AH4.GPP_CLK1P -16,-8; AH5.GPP_CLK1N -15,-8; AH6.VDDCR_CPU -14,-8; AH7.GPP_CLK2P -13,-8; AH8.GPP_CLK2N -12,-8; AH9.VDDCR_CPU -11,-8; AH10.VSS -10,-8; AH11.VDDCR_CPU -9,-8; AH12.VSS -8,-8; AH13.VDDCR_CPU -7,-8; AH14.VSS -6,-8; AH15.VDDCR_CPU -5,-8; AH16.VSS -4,-8; AH17.VDDCR_CPU -3,-8; AH18.VSS -2,-8; AH19.VDDCR_CPU -1,-8; AH20.VSS 0,-8; AH21.VDDCR_CPU 1,-8; AH22.VSS 2,-8; AH23.VDDCR_CPU 3,-8; AH24.VSS 4,-8; AH25.VDDCR_CPU 5,-8; AH26.VSS 6,-8; AH27.VDDCR_CPU 7,-8; AH28.VSS 8,-8; AH29.VSS 9,-8; AH30.VSS 10,-8; AH31.MA_DATA[36] 11,-8; AH32.MA_DATA[37] 12,-8; AH33.VSS 13,-8; AH34.MA_DATA[32] 14,-8; AH35.RSVD 15,-8; AH36.MB0_ODT[1] 16,-8; AH37.MB_ADD_17 17,-8; AH38.MB1_ODT[1] 18,-8; AH39.VDDIO_MEM_S3 19,-8; AJ2.VDDCR_CPU -18,-9; AJ3.USB0_ZVSS -17,-9; AJ4.USB_SS_ZVSS -16,-9; AJ5.VSS -15,-9; AJ6.GPP_CLK3P -14,-9; AJ7.GPP_CLK3N -13,-9; AJ8.VSS -12,-9; AJ9.VSS -11,-9; AJ10.VDDCR_CPU -10,-9; AJ11.VSS -9,-9; AJ12.VDDCR_CPU -8,-9; AJ13.VSS -7,-9; AJ14.VDDCR_CPU -6,-9; AJ15.VDD_18_S5 -5,-9; AJ16.VDDP_S5 -4,-9; AJ17.VDDP_S5 -3,-9; AJ18.VDDCR_SOC_S5 -2,-9; AJ19.VDD_33_S5 -1,-9; AJ20.VDD_18 0,-9; AJ21.VDD_33 1,-9; AJ22.VDDCR_CPU 2,-9; AJ23.VSS 3,-9; AJ24.VDDCR_CPU 4,-9; AJ25.VSS 5,-9; AJ26.VSS 6,-9; AJ27.VSS 7,-9; AJ28.VSS 8,-9; AJ29.VSS 9,-9; AJ30.MA_DATA[33] 10,-9; AJ31.MA_DM[4] 11,-9; AJ32.VSS 12,-9; AJ33.MA_DQS_H[4] 13,-9; AJ34.MA_DQS_L[4] 14,-9; AJ35.VSS 15,-9; AJ36.VSS 16,-9; AJ37.MA_ZVSS 17,-9; AJ38.VSS 18,-9; AJ39.MB_ZVSS 19,-9; AK1.VSS -19,-10; AK2.SDA1/I2C3_SDA/AGPIO20 -18,-10; AK3.SCL1/I2C3_SCL/AGPIO19 -17,-10; AK4.VSS -16,-10; AK5.USB3_ZVSS -15,-10; AK6.USB2_ZVSS -14,-10; AK7.VDDCR_CPU -13,-10; AK8.USB_SS_ZVDDP -12,-10; AK9.VDDCR_CPU -11,-10; AK10.VSS -10,-10; AK11.VDDCR_CPU -9,-10; AK12.VSS -8,-10; AK13.VDDCR_CPU -7,-10; AK14.VSS -6,-10; AK15.VDD_18_S5 -5,-10; AK18.VDDCR_SOC_S5 -2,-10; AK19.VDD_33_S5 -1,-10; AK20.VDD_18 0,-10; AK21.VDD_33 1,-10; AK22.VSS 2,-10; AK25.VSS 5,-10; AK26.MA_DATA[57] 6,-10; AK27.MA_DATA[56] 7,-10; AK28.VSS 8,-10; AK29.MA_DATA[49] 9,-10; AK30.MA_DATA[34] 10,-10; AK31.VSS 11,-10; AK32.MA_DATA[39] 12,-10; AK33.MA_DATA[38] 13,-10; AK34.RSVD 14,-10; AK35.VSS 15,-10; AK36.MB_DATA[37] 16,-10; AK37.VSS 17,-10; AK38.MB_DATA[36] 18,-10; AK39.MB_DATA[32] 19,-10; AL2.LPC_PME_L/AGPIO22 -18,-11; AL3.VDDCR_CPU -17,-11; AL4.TEST46[13] -16,-11; AL5.WAKE_L/AGPIO2 -15,-11; AL6.VDDCR_CPU -14,-11; AL7.PCIE_RST_L/EGPIO26 -13,-11; AL8.AM4R1 -12,-11; AL9.VSS -11,-11; AL10.VDDCR_CPU -10,-11; AL11.VSS -9,-11; AL12.VDDCR_CPU -8,-11; AL13.P_GPP_TXP[2]/SATA_TX0P -7,-11; AL14.VDDCR_CPU -6,-11; AL15.VDDBT_RTC_G -5,-11; AL16.RSVD -4,-11; AL17.RSVD -3,-11; AL18.RSVD -2,-11; AL19.RSVD -1,-11; AL20.RSVD 0,-11; AL21.RSVD 1,-11; AL22.VDDP_SENSE 2,-11; AL23.CLK_REQ3_L/SATA_IS1_L/SATA_ZP1_L/EGPIO131 3,-11; AL24.VSS 4,-11; AL25.MA_DATA[62] 5,-11; AL26.MA_DM[7] 6,-11; AL27.VSS 7,-11; AL28.MA_DATA[51] 8,-11; AL29.MA_DM[6] 9,-11; AL30.VSS 10,-11; AL31.MA_DATA[45] 11,-11; AL32.MA_DATA[44] 12,-11; AL33.VSS 13,-11; AL34.MA_DATA[35] 14,-11; AL35.VSS 15,-11; AL36.VSS 16,-11; AL37.MB_DATA[33] 17,-11; AL38.MB_DM[4] 18,-11; AL39.VSS 19,-11; AM2.VDDCR_CPU -18,-12; AM3.PWR_GOOD -17,-12; AM4.SYS_RESET_L/AGPIO1 -16,-12; AM5.VSS -15,-12; AM6.TEST0 -14,-12; AM7.TEST1/TMS -13,-12; AM8.VDDCR_CPU -12,-12; AM9.P_GPP_RXP[1] -11,-12; AM10.P_GPP_RXN[1] -10,-12; AM11.VSS -9,-12; AM12.RSVD -8,-12; AM13.P_GPP_TXN[2]/SATA_TX0N -7,-12; AM14.VSS -6,-12; AM15.VDDIO_AUDIO -5,-12; AM16.RSVD -4,-12; AM17.RSVD -3,-12; AM18.VDDP -2,-12; AM19.VDDP -1,-12; AM20.VDDP 0,-12; AM21.RSVD 1,-12; AM22.SATA_ACT_L/AGPIO130 2,-12; AM23.VSS_SENSE_B 3,-12; AM24.CORETYPE[0] 4,-12; AM25.MA_DATA[63] 5,-12; AM26.VSS 6,-12; AM27.MA_DATA[61] 7,-12; AM28.MA_DATA[50] 8,-12; AM29.VSS 9,-12; AM30.MA_DATA[52] 10,-12; AM31.MA_DM[5] 11,-12; AM32.VSS 12,-12; AM33.MA_DATA[41] 13,-12; AM34.MA_DATA[40] 14,-12; AM35.VSS 15,-12; AM36.MB_DQS_L[4] 16,-12; AM37.MB_DQS_H[4] 17,-12; AM38.VSS 18,-12; AM39.MB_DATA[38] 19,-12; AN2.AGPIO9/SGPIO0_DATAOUT -18,-13; AN3.AGPIO23/SGPIO0_LOAD -17,-13; AN4.VSS -16,-13; AN5.PWR_BTN_L/AGPIO0 -15,-13; AN6.USB1_ZVSS -14,-13; AN7.VDDCR_CPU -13,-13; AN8.AGPIO6 -12,-13; AN9.CORETYPE[1] -11,-13; AN10.VDDCR_CPU -10,-13; AN11.P_GPP_RXN[3]/SATA_RX1N -9,-13; AN12.RSVD -8,-13; AN13.VDDCR_CPU -7,-13; AN14.P_GPP_TXP[3]/SATA_TX1P -6,-13; AN15.RSVD -5,-13; AN16.RSVD -4,-13; AN17.RSVD -3,-13; AN18.VDDP -2,-13; AN19.VDDP -1,-13; AN20.VDDP 0,-13; AN21.RSVD 1,-13; AN22.VSS 2,-13; AN23.FANIN0/AGPIO84 3,-13; AN24.ESPI_RESET_L/KBRST_L 4,-13; AN25.VSS 5,-13; AN26.MA_DQS_L[7] 6,-13; AN27.MA_DATA[60] 7,-13; AN28.VSS 8,-13; AN29.MA_DQS_L[6] 9,-13; AN30.MA_DATA[53] 10,-13; AN31.VSS 11,-13; AN32.MA_DQS_H[5] 12,-13; AN33.MA_DQS_L[5] 13,-13; AN34.VSS 14,-13; AN35.VSS 15,-13; AN36.MB_DATA[34] 16,-13; AN37.VSS 17,-13; AN38.MB_DATA[39] 18,-13; AN39.MB_DATA[35] 19,-13; AP2.SLP_S5_L -18,-14; AP3.VDDCR_CPU -17,-14; AP4.S5_MUX_CTRL/EGPIO42 -16,-14; AP5.RSMRST_L -15,-14; AP6.VSS -14,-14; AP7.AGPIO8 -13,-14; AP8.RTCCLK -12,-14; AP9.VDDCR_CPU -11,-14; AP10.P_GPP_RXN[2]/SATA_RX0N -10,-14; AP11.P_GPP_RXP[3]/SATA_RX1P -9,-14; AP12.VDDCR_CPU -8,-14; AP13.P_GPP_TXP[1] -7,-14; AP14.P_GPP_TXN[3]/SATA_TX1N -6,-14; AP15.RSVD -5,-14; AP16.RSVD -4,-14; AP17.RSVD -3,-14; AP18.VDDP -2,-14; AP19.VDDP -1,-14; AP20.VDDP 0,-14; AP21.RSVD 1,-14; AP22.AGPIO5/DEVSLP0 2,-14; AP23.FANOUT0/AGPIO85 3,-14; AP24.VSS 4,-14; AP25.MA_DATA[58] 5,-14; AP26.MA_DQS_H[7] 6,-14; AP27.VSS 7,-14; AP28.MA_DATA[54] 8,-14; AP29.MA_DQS_H[6] 9,-14; AP30.VSS 10,-14; AP31.MA_DATA[42] 11,-14; AP32.MA_DATA[47] 12,-14; AP33.VSS 13,-14; AP34.MA_DATA[46] 14,-14; AP35.VSS 15,-14; AP36.VSS 16,-14; AP37.MB_DATA[44] 17,-14; AP38.MB_DATA[45] 18,-14; AP39.VSS 19,-14; AR2.VDDCR_CPU -18,-15; AR3.S0A3_GPIO/AGPIO10/SGPIO0_CLK -17,-15; AR4.AGPIO40/SGPIO0_DATAIN -16,-15; AR5.VSS -15,-15; AR6.AGPIO4 -14,-15; AR7.48M_OSC -13,-15; AR8.VSS -12,-15; AR9.P_GPP_RXP[0] -11,-15; AR10.P_GPP_RXP[2]/SATA_RX0P -10,-15; AR11.VSS -9,-15; AR12.P_GPP_TXN[0] -8,-15; AR13.P_GPP_TXN[1] -7,-15; AR14.VSS -6,-15; AR15.RSVD -5,-15; AR16.RSVD -4,-15; AR17.VSS -3,-15; AR18.RSVD -2,-15; AR19.RSVD -1,-15; AR20.RSVD 0,-15; AR21.RSVD 1,-15; AR22.CLK_REQG_L/OSCIN/EGPIO132 2,-15; AR23.VSS 3,-15; AR24.RSVD 4,-15; AR25.MA_DATA[59] 5,-15; AR26.VSS 6,-15; AR27.VSS 7,-15; AR28.MA_DATA[55] 8,-15; AR29.VSS 9,-15; AR30.VSS 10,-15; AR31.MA_DATA[48] 11,-15; AR32.VSS 12,-15; AR33.MA_DATA[43] 13,-15; AR34.VSS 14,-15; AR35.VSS 15,-15; AR36.MB_DATA[40] 16,-15; AR37.MB_DATA[41] 17,-15; AR38.VSS 18,-15; AR39.MB_DM[5] 19,-15; AT2.SLP_S3_L -18,-16; AT3.TEST2 -17,-16; AT4.VDDCR_CPU -16,-16; AT5.BLINK/AGPIO11 -15,-16; AT6.AGPIO3 -14,-16; AT7.VSS -13,-16; AT8.P0B_ZVSS -12,-16; AT9.P_GPP_RXN[0] -11,-16; AT10.VSS -10,-16; AT11.USB_ZVSS -9,-16; AT12.P_GPP_TXP[0] -8,-16; AT13.VSS -7,-16; AT14.EGPIO100 -6,-16; AT15.ESPI_ALERT_L/LDRQ0_L/EGPIO108 -5,-16; AT16.VSS -4,-16; AT17.SPI_CS1_L/EGPIO118 -3,-16; AT18.EGPIO70 -2,-16; AT19.RSVD -1,-16; AT20.LAD3/EGPIO107 0,-16; AT21.LAD2/EGPIO106 1,-16; AT22.VSS 2,-16; AT23.CLK_REQ0_L/SATA_IS0_L/SATA_ZP0_L/AGPIO92 3,-16; AT24.CLK_REQ2_L/AGPIO116 4,-16; AT25.RSVD 5,-16; AT26.VSS 6,-16; AT27.VSS 7,-16; AT28.VSS 8,-16; AT29.VSS 9,-16; AT30.RSVD 10,-16; AT31.VSS 11,-16; AT32.VSS 12,-16; AT33.VSS 13,-16; AT34.VSS 14,-16; AT35.MB_DM[6] 15,-16; AT36.MB_DATA[46] 16,-16; AT37.VSS 17,-16; AT38.MB_DQS_H[5] 18,-16; AT39.MB_DQS_L[5] 19,-16; AU2.AZ_SYNC -18,-17; AU3.VDDCR_CPU -17,-17; AU4.AZ_SDOUT -16,-17; AU5.AZ_SDIN1 -15,-17; AU6.VDDCR_CPU -14,-17; AU7.USB_HSD0P -13,-17; AU8.USB_HSD0N -12,-17; AU9.VDDCR_CPU -11,-17; AU10.USB_HSD2P -10,-17; AU11.USB_HSD2N -9,-17; AU12.VDDCR_CPU -8,-17; AU13.EGPIO98 -7,-17; AU14.SPI_DI/ESPI_DAT1/EGPIO120 -6,-17; AU15.VDDCR_CPU -5,-17; AU16.SPI_DO/ESPI_DAT0/EGPIO121 -4,-17; AU17.SPI_TPM_CS_L/AGPIO76 -3,-17; AU18.VSS -2,-17; AU19.LPCCLK1/EGPIO75 -1,-17; AU20.LPCCLK0/EGPIO74 0,-17; AU21.VSS 1,-17; AU22.LPC_RST_L 2,-17; AU23.GENINT2_L/AGPIO90 3,-17; AU24.VSS 4,-17; AU25.SCL0/I2C2_SCL/EGPIO113 5,-17; AU26.VSS 6,-17; AU27.VSS 7,-17; AU28.MB_DQS_H[7] 8,-17; AU29.MB_DQS_L[7] 9,-17; AU30.VSS 10,-17; AU31.MB_DATA[61] 11,-17; AU32.MB_DATA[51] 12,-17; AU33.VSS 13,-17; AU34.MB_DQS_H[6] 14,-17; AU35.MB_DATA[49] 15,-17; AU36.VSS 16,-17; AU37.MB_DATA[42] 17,-17; AU38.MB_DATA[47] 18,-17; AU39.VSS 19,-17; AV3.AZ_SDIN0 -17,-18; AV4.AZ_SDIN2 -16,-18; AV5.VDDCR_CPU -15,-18; AV6.SATA_ZVSS -14,-18; AV7.SATA_ZVDDP -13,-18; AV8.VDDCR_CPU -12,-18; AV9.USB_HSD3P -11,-18; AV10.USB_HSD3N -10,-18; AV11.VDDCR_CPU -9,-18; AV12.EGPIO96 -8,-18; AV13.EGPIO99 -7,-18; AV14.VDDCR_CPU -6,-18; AV15.SPI_HOLD_L/ESPI_DAT3/EGPIO133 -5,-18; AV16.SPI_WP_L/ESPI_DAT2/EGPIO122 -4,-18; AV17.VSS -3,-18; AV18.LPC_PD_L/AGPIO21 -2,-18; AV19.LPC_CLKRUN_L/AGPIO88 -1,-18; AV20.VSS 0,-18; AV21.LAD1/EGPIO105 1,-18; AV22.GENINT1_L/AGPIO89 2,-18; AV23.VSS 3,-18; AV24.CLK_REQ1_L/AGPIO115 4,-18; AV25.SDA0/I2C2_SDA/EGPIO114 5,-18; AV26.VSS 6,-18; AV27.MB_DATA[63] 7,-18; AV28.MB_DATA[62] 8,-18; AV29.VSS 9,-18; AV30.MB_DATA[57] 10,-18; AV31.MB_DATA[60] 11,-18; AV32.VSS 12,-18; AV33.MB_DATA[55] 13,-18; AV34.MB_DQS_L[6] 14,-18; AV35.VSS 15,-18; AV36.MB_DATA[52] 16,-18; AV37.MB_DATA[43] 17,-18; AV38.VSS 18,-18; AW4.VSS -16,-19; AW5.X32K_X1 -15,-19; AW6.X32K_X2 -14,-19; AW7.VSS -13,-19; AW8.USB_HSD1P -12,-19; AW9.USB_HSD1N -11,-19; AW10.VSS -10,-19; AW11.EGPIO95 -9,-19; AW12.EGPIO97 -8,-19; AW13.VSS -7,-19; AW14.SPI_CLK/ESPI_CLK/EGPIO117 -6,-19; AW15.SPI_CS2_L/ESPI_CS_L/EGPIO119 -5,-19; AW16.VSS -4,-19; AW17.AGPIO86 -3,-19; AW18.LFRAME_L/EGPIO109 -2,-19; AW19.VSS -1,-19; AW20.LAD0/EGPIO104 0,-19; AW21.SERIRQ/AGPIO87 1,-19; AW22.VSS 2,-19; AW23.SPKR/AGPIO91 3,-19; AW24.RSVD 4,-19; AW25.VSS 5,-19; AW26.MB_DATA[59] 6,-19; AW27.MB_DATA[58] 7,-19; AW28.VSS 8,-19; AW29.MB_DM[7] 9,-19; AW30.MB_DATA[56] 10,-19; AW31.VSS 11,-19; AW32.MB_DATA[50] 12,-19; AW33.MB_DATA[54] 13,-19; AW34.VSS 14,-19; AW35.MB_DATA[48] 15,-19; AW36.MB_DATA[53] 16,-19; AW37.VSS 17,-19; B4.DP0_TXP[2] -16,18; B5.VDDCR_SOC -15,18; B6.DP2_TXP[0] -14,18; B7.DP2_TXN[0] -13,18; B8.VDDCR_SOC -12,18; B9.DP2_TXP[3] -11,18; B10.DP2_TXN[3] -10,18; B11.VDDCR_SOC -9,18; B12.TEST15 -8,18; B13.TRST_L -7,18; B14.VDDCR_SOC -6,18; B15.TMS -5,18; B16.RESET_L -4,18; B17.VDDCR_SOC -3,18; B18.SIC -2,18; B19.VSS -1,18; B20.VDDCR_SOC 0,18; B21.MB_DATA[1] 1,18; B22.MB_DQS_H[0] 2,18; B23.VSS 3,18; B24.MB_DATA[2] 4,18; B25.MB_DATA[13] 5,18; B26.VSS 6,18; B27.MB_DQS_L[1] 7,18; B28.MB_DATA[15] 8,18; B29.VSS 9,18; B30.MB_DATA[20] 10,18; B31.MB_DATA[17] 11,18; B32.VSS 12,18; B33.MB_DATA[22] 13,18; B34.MB_DATA[18] 14,18; B35.VSS 15,18; B36.MB_DATA[24] 16,18; B37.MB_DQS_H[3] 17,18; B38.MB_DATA[30] 18,18; C2.DP0_TXN[0] -18,17; C3.DP0_TXP[1] -17,17; C4.VDDCR_SOC -16,17; C5.DP0_TXP[3] -15,17; C6.DP0_TXN[3] -14,17; C7.VDDCR_SOC -13,17; C8.DP2_TXP[2] -12,17; C9.DP2_TXN[2] -11,17; C10.VDDCR_SOC -10,17; C11.TEST16 -9,17; C12.TEST14 -8,17; C13.VDDCR_SOC -7,17; C14.TDO -6,17; C15.TCK -5,17; C16.VDDCR_SOC -4,17; C17.SVD -3,17; C18.SID -2,17; C19.VDDCR_SOC -1,17; C20.MB_DATA[5] 0,17; C21.MB_DM[0] 1,17; C22.VSS 2,17; C23.MB_DATA[7] 3,17; C24.MB_DATA[3] 4,17; C25.VSS 5,17; C26.MB_DATA[9] 6,17; C27.MB_DQS_H[1] 7,17; C28.VSS 8,17; C29.MB_DATA[11] 9,17; C30.MB_DATA[21] 10,17; C31.VSS 11,17; C32.MB_DQS_L[2] 12,17; C33.MB_DQS_H[2] 13,17; C34.VSS 14,17; C35.MB_DATA[19] 15,17; C36.MB_DATA[29] 16,17; C37.VSS 17,17; C38.MB_DATA[31] 18,17; C39.MB_DATA[26] 19,17; D2.DP0_TXP[0] -18,16; D3.VDDCR_SOC -17,16; D4.DP1_TXP[0] -16,16; D5.DP1_TXN[0] -15,16; D6.VSS -14,16; D7.DP1_TXP[1] -13,16; D8.DP1_TXN[1] -12,16; D9.VSS -11,16; D10.DP1_HPD -10,16; D11.TEST17 -9,16; D12.VSS -8,16; D13.TEST6 -7,16; D14.DBREQ_L -6,16; D15.VSS -5,16; D16.ALERT_L -4,16; D17.SVC -3,16; D18.VSS -2,16; D19.VSS -1,16; D20.MB_DATA[0] 0,16; D21.VSS 1,16; D22.VSS 2,16; D23.VSS 3,16; D24.VSS 4,16; D25.VSS 5,16; D26.MB_DM[1] 6,16; D27.VSS 7,16; D28.RSVD 8,16; D29.VSS 9,16; D30.VSS 10,16; D31.VSS 11,16; D32.VSS 12,16; D33.VSS 13,16; D34.VSS 14,16; D35.VSS 15,16; D36.VSS 16,16; D37.MB_DM[3] 17,16; D38.MB_DATA[27] 18,16; D39.VSS 19,16; E2.VDDCR_SOC -18,15; E3.P_GFX_TXP[1] -17,15; E4.VSS -16,15; E5.VSS -15,15; E6.TEST28_H -14,15; E7.TEST28_L -13,15; E8.VSS -12,15; E9.DP1_TXP[3] -11,15; E10.DP2_HPD -10,15; E11.VSS -9,15; E12.DP_AUX_ZVSS -8,15; E13.DBRDY -7,15; E14.VSS -6,15; E15.VDDCR_SOC_SENSE -5,15; E16.PWROK -4,15; E17.VSS -3,15; E18.MA_DATA[0] -2,15; E19.RSVD -1,15; E20.VSS 0,15; E21.VSS 1,15; E22.RSVD 2,15; E23.VSS 3,15; E24.MA_DATA[10] 4,15; E25.RSVD 5,15; E26.VSS 6,15; E27.VSS 7,15; E28.MA_DATA[22] 8,15; E29.VSS 9,15; E30.MA_DQS_L[3] 10,15; E31.MA_DATA[30] 11,15; E32.VSS 12,15; E33.MA_CHECK[4] 13,15; E34.MA_CHECK[5] 14,15; E35.VSS 15,15; E36.MB_DATA[25] 16,15; E37.MB_CHECK[4] 17,15; E38.VSS 18,15; E39.MB_CHECK[5] 19,15; F2.P_GFX_TXP[2] -18,14; F3.P_GFX_TXN[1] -17,14; F4.VSS -16,14; F5.P_GFX_RXN[0] -15,14; F6.P_GFX_RXP[0] -14,14; F7.VDDCR_SOC -13,14; F8.DP1_TXP[2] -12,14; F9.DP1_TXN[3] -11,14; F10.VDDCR_SOC -10,14; F11.DP1_AUXP -9,14; F12.DP_ZVSS -8,14; F13.VDDCR_SOC -7,14; F14.VDDCR_CPU_SENSE -6,14; F15.VSS_SENSE_A -5,14; F16.VDDCR_SOC -4,14; F17.VSS -3,14; F18.MA_DATA[5] -2,14; F19.VSS -1,14; F20.MA_DATA[7] 0,14; F21.MA_DATA[12] 1,14; F22.VSS 2,14; F23.MA_DQS_H[1] 3,14; F24.MA_DATA[15] 4,14; F25.VSS 5,14; F26.MA_DQS_L[2] 6,14; F27.MA_DQS_H[2] 7,14; F28.VSS 8,14; F29.MA_DATA[24] 9,14; F30.MA_DQS_H[3] 10,14; F31.VSS 11,14; F32.MA_DATA[27] 12,14; F33.MA_CHECK[0] 13,14; F34.VSS 14,14; F35.VSS 15,14; F36.MB_CHECK[1] 16,14; F37.VSS 17,14; F38.MB_CHECK[0] 18,14; F39.MB_DM[8] 19,14; G2.P_GFX_TXN[2] -18,13; G3.VDDCR_SOC -17,13; G4.P_GFX_RXN[1] -16,13; G5.P_GFX_RXP[1] -15,13; G6.VDDCR_SOC -14,13; G7.VSS -13,13; G8.DP1_TXN[2] -12,13; G9.VDDCR_SOC -11,13; G10.DP0_AUXP -10,13; G11.DP1_AUXN -9,13; G12.VDDCR_SOC -8,13; G13.DP_BLON -7,13; G14.VDDIO_MEM_S3_SENSE -6,13; G15.VDDCR_SOC -5,13; G16.TEST18 -4,13; G17.RSVD -3,13; G18.VDDCR_SOC -2,13; G19.MA_DQS_L[0] -1,13; G20.MA_DATA[6] 0,13; G21.VSS 1,13; G22.MA_DATA[9] 2,13; G23.MA_DQS_L[1] 3,13; G24.VSS 4,13; G25.MA_DATA[21] 5,13; G26.MA_DM[2] 6,13; G27.VSS 7,13; G28.MA_DATA[18] 8,13; G29.MA_DATA[29] 9,13; G30.VSS 10,13; G31.MA_DATA[31] 11,13; G32.MA_CHECK[1] 12,13; G33.VSS 13,13; G34.MA_DM[8] 14,13; G35.VSS 15,13; G36.VSS 16,13; G37.MB_DQS_L[8] 17,13; G38.MB_DQS_H[8] 18,13; G39.VSS 19,13; H2.VDDCR_SOC -18,12; H3.P_GFX_TXP[4] -17,12; H4.VSS -16,12; H5.VSS -15,12; H6.P_GFX_RXN[2] -14,12; H7.P_GFX_RXP[2] -13,12; H8.VSS -12,12; H9.DP0_HPD -11,12; H10.DP0_AUXN -10,12; H11.VSS -9,12; H12.DP_VARYBL -8,12; H13.DP_DIGON -7,12; H14.VSS -6,12; H15.PROCHOT_L -5,12; H16.TEST19 -4,12; H17.VSS -3,12; H18.MA_DATA[4] -2,12; H19.MA_DQS_H[0] -1,12; H20.VSS 0,12; H21.MA_DATA[3] 1,12; H22.MA_DATA[8] 2,12; H23.VSS 3,12; H24.MA_DATA[14] 4,12; H25.MA_DATA[20] 5,12; H26.VSS 6,12; H27.MA_DATA[23] 7,12; H28.MA_DATA[19] 8,12; H29.VSS 9,12; H30.MA_DM[3] 10,12; H31.MA_DATA[26] 11,12; H32.VSS 12,12; H33.MA_DQS_L[8] 13,12; H34.MA_DQS_H[8] 14,12; H35.VSS 15,12; H36.MB_CHECK[6] 16,12; H37.MB_CHECK[7] 17,12; H38.VSS 18,12; H39.MB_CHECK[2] 19,12; J2.P-GFX_TXP[5] -18,11; J3.P_GFX_TXN[4] -17,11; J4.VSS -16,11; J5.P_GFX_RXN[3] -15,11; J6.P_GFX_RXP[3] -14,11; J7.VDDCR_SOC -13,11; J8.VSS -12,11; J9.VSS -11,11; J10.VDDCR_SOC -10,11; J11.VSS -9,11; J12.VDDCR_SOC -8,11; J13.VSS -7,11; J14.VDDCR_SOC -6,11; J15.VSS -5,11; J16.VDDCR_SOC -4,11; J17.VSS -3,11; J18.MA_DATA[1] -2,11; J19.VSS -1,11; J20.MA_DATA[2] 0,11; J21.MA_DATA[13] 1,11; J22.VSS 2,11; J23.MA_DM[1] 3,11; J24.MA_DATA[11] 4,11; J25.VSS 5,11; J26.MA_DATA[16] 6,11; J27.MA_DATA[17] 7,11; J28.VSS 8,11; J29.MA_DATA[28] 9,11; J30.MA_DATA[25] 10,11; J31.VSS 11,11; J32.MA_CHECK[6] 12,11; J33.MA_CHECK[7] 13,11; J34.VSS 14,11; J35.VSS 15,11; J36.RSVD 16,11; J37.VSS 17,11; J38.RSVD 18,11; J39.MB_CHECK[3] 19,11; K1.P_GFX_TXP[6] -19,10; K2.P_GFX_TXN[5] -18,10; K3.VDDCR_SOC -17,10; K4.P_GFX_RXN[5] -16,10; K5.P_GFX_RXP[5] -15,10; K6.VDDCR_SOC -14,10; K7.P_GFX_RXN[4] -13,10; K8.P_GFX_RXP[4] -12,10; K9.VDDCR_SOC -11,10; K10.VSS -10,10; K11.VDDCR_SOC -9,10; K12.VSS -8,10; K13.VDDCR_SOC -7,10; K14.DP_STEREOSYNC -6,10; K15.VDDCR_SOC -5,10; K18.VSS -2,10; K19.MA_DM[0] -1,10; K20.VSS 0,10; K21.VSS 1,10; K22.VSS 2,10; K23.VSS 3,10; K26.VSS 6,10; K27.VSS 7,10; K28.VSS 8,10; K29.VSS 9,10; K30.VSS 10,10; K31.MA_CHECK[2] 11,10; K32.MA_CHECK[3] 12,10; K33.VSS 13,10; K34.RSVD 14,10; K35.MB_RESET_L 15,10; K36.VDDIO_MEM_S3 16,10; K37.MB0_CKE[1] 17,10; K38.RSVD 18,10; K39.VDDIO_MEM_S3 19,10; L2.VDDCR_SOC -18,9; L3.P_GFX_TXP[7] -17,9; L4.VSS -16,9; L5.VSS -15,9; L6.P_GFX_RXN[6] -14,9; L7.P_GFX_RXP[6] -13,9; L8.VSS -12,9; L9.VSS -11,9; L10.VDDCR_SOC -10,9; L11.VSS -9,9; L12.VDDCR_SOC -8,9; L13.VSS -7,9; L14.VDDCR_SOC -6,9; L15.VSS -5,9; L16.VDDCR_SOC -4,9; L17.VSS -3,9; L18.VDDCR_SOC -2,9; L19.VSS -1,9; L20.VDDCR_SOC 0,9; L21.VSS 1,9; L22.VDDCR_SOC 2,9; L23.TEST4 3,9; L24.VDDCR_SOC 4,9; L25.VSS 5,9; L26.VDDCR_SOC 6,9; L27.VSS 7,9; L28.VSS 8,9; L29.VSS 9,9; L30.VSS 10,9; L31.VSS 11,9; L32.VDDIO_MEM_S3 12,9; L33.MA_RESET_L 13,9; L34.MA1_CKE[1] 14,9; L35.VDDIO_MEM_S3 15,9; L36.MB1_CKE[1] 16,9; L37.MB0_CKE[0] 17,9; L38.VDDIO_MEM_S3 18,9; L39.MB1_CKE[0] 19,9; M2.P_GFX_TXP[8] -18,8; M3.P_GFX_TXN[7] -17,8; M4.VSS -16,8; M5.P_GFX_RXN[7] -15,8; M6.P_GFX_RXP[7] -14,8; M7.VDDCR_CPU -13,8; M8.VSS -12,8; M9.VDDCR_SOC -11,8; M10.VSS -10,8; M11.VDDCR_SOC -9,8; M12.VSS -8,8; M13.VDDCR_SOC -7,8; M14.VSS -6,8; M15.VDDCR_SOC -5,8; M16.VSS -4,8; M17.VDDCR_SOC -3,8; M18.VSS -2,8; M19.VDDCR_SOC -1,8; M20.VSS 0,8; M21.VDDCR_SOC 1,8; M22.TEST5 2,8; M23.VDDCR_SOC 3,8; M24.VSS 4,8; M25.VDDCR_SOC 5,8; M26.VSS 6,8; M27.VSS 7,8; M28.VSS 8,8; M29.VDDIO_MEM_S3 9,8; M30.MA0_CKE[1] 10,8; M31.VDDIO_MEM_S3 11,8; M32.MA0_CKE[0] 12,8; M33.MA1_CKE[0] 13,8; M34.VDDIO_MEM_S3 14,8; M35.MA_ACT_L 15,8; M36.MB_BG[0] 16,8; M37.VDDIO_MEM_S3 17,8; M38.MB_ACT_L 18,8; M39.MB_BG[1] 19,8; N2.P_GFX_TXN[8] -18,7; N3.VDDCR_CPU -17,7; N4.P_GFX_RXN[9] -16,7; N5.P_GFX_RXP[9] -15,7; N6.VDDCR_CPU -14,7; N7.P_GFX_RXN[8] -13,7; N8.P_GFX_RXP[8] -12,7; N9.VSS -11,7; N10.VDDCR_SOC -10,7; N11.VSS -9,7; N12.VDDCR_SOC -8,7; N13.VSS -7,7; N14.VDDCR_SOC -6,7; N15.VSS -5,7; N16.VDDCR_SOC -4,7; N17.VSS -3,7; N18.VDDCR_SOC -2,7; N19.VSS -1,7; N20.VDDCR_SOC 0,7; N21.VSS 1,7; N22.VDDCR_SOC 2,7; N23.VSS 3,7; N24.VDDCR_SOC 4,7; N25.VSS 5,7; N26.VDDCR_SOC 6,7; N27.VSS 7,7; N28.VDDIO_MEM_S3 8,7; N29.VSS 9,7; N30.VDDIO_MEM_S3 10,7; N31.MA_BG[0] 11,7; N32.MA_BG[1] 12,7; N33.VDDIO_MEM_S3 13,7; N34.MA_ALERT_L 14,7; N35.MA_ADD[12] 15,7; N36.VDDIO_MEM_S3 16,7; N37.MB_ALERT_L 17,7; N38.MB_ADD[12] 18,7; N39.VDDIO_MEM_S3 19,7; P1.P_GFX_TXN[9] -19,6; P2.VDDCR_CPU -18,6; P3.P_GFX_TXP[10] -17,6; P4.VSS -16,6; P5.VSS -15,6; P6.P_GFX_RXN[10] -14,6; P7.P_GFX_RXP[10] -13,6; P8.VSS -12,6; P9.VDDCR_SOC -11,6; P10.VSS -10,6; P11.VDDCR_SOC -9,6; P12.VSS -8,6; P13.VDDCR_SOC -7,6; P27.VDDIO_MEM_S3 7,6; P28.TEST47 8,6; P29.VDDIO_MEM_S3 9,6; P30.MA_ADD[8] 10,6; P31.MA_ADD[9] 11,6; P32.VDDIO_MEM_S3 12,6; P33.MA_ADD[11] 13,6; P34.MA_ADD[7] 14,6; P35.VDDIO_MEM_S3 15,6; P36.MB_ADD[9] 16,6; P37.MB_ADD[11] 17,6; P38.VDDIO_MEM_S3 18,6; P39.MB_ADD[7] 19,6; R1.VSS -19,5; R2.P_GFX_TXP[11] -18,5; R3.P_GFX_TXN[10] -17,5; R4.VSS -16,5; R5.P_GFX_RXN[11] -15,5; R6.P_GFX_RXP[11] -14,5; R7.VDDCR_CPU -13,5; R8.VSS -12,5; R9.VSS -11,5; R10.VDDCR-SOC -10,5; R11.VSS -9,5; R12.VDDCR_SOC -8,5; R13.VSS -7,5; R27.VSS 7,5; R28.VDDIO_MEM_S3 8,5; R29.VSS 9,5; R30.MA_ADD[4] 10,5; R31.VDDIO_MEM_S3 11,5; R32.MA_ADD[6] 12,5; R33.MA_ADD[5] 13,5; R34.VDDIO_MEM_S3 14,5; R35.RSVD 15,5; R36.MB_ADD[6] 16,5; R37.VDDIO_MEM_S3 17,5; R38.MB_ADD[8] 18,5; R39.MB_ADD[5] 19,5; T1.P_GFX_TXP[12] -19,4; T2.P_GFX_TXN[11] -18,4; T3.VDDCR_CPU -17,4; T4.P_GFX_RXP[13] -16,4; T5.P_GFX_RXN[13] -15,4; T6.VDDCR_CPU -14,4; T7.P_GFX_RXN[12] -13,4; T8.P_GFX_RXP[12] -12,4; T9.VDDCR_CPU -11,4; T10.VSS -10,4; T11.VDDCR_SOC -9,4; T12.VSS -8,4; T13.VDDCR_SOC -7,4; T27.VDDIO_MEM_S3 7,4; T28.VSS 8,4; T29.VDDIO_MEM_S3 9,4; T30.VSS 10,4; T31.MA_ADD[3] 11,4; T32.MA_ADD[1] 12,4; T33.VDDIO_MEM_S3 13,4; T34.MA_CLK_H[0] 14,4; T35.MA_ADD[2] 15,4; T36.VDDIO_MEM_S3 16,4; T37.MB_ADD[4] 17,4; T38.MB_ADD[3] 18,4; T39.VDDIO_MEM_S3 19,4; U1.P_GFX_TXN[12] -19,3; U2.VDDCR_CPU -18,3; U3.P_GFX_TXP[13] -17,3; U4.VSS -16,3; U5.VSS -15,3; U6.P_GFX_RXN[14] -14,3; U7.P_GFX_RXP[14] -13,3; U8.VSS -12,3; U9.VSS -11,3; U10.VDDCR_CPU -10,3; U11.VSS -9,3; U12.VDDCR_SOC -8,3; U13.VSS -7,3; U27.VSS 7,3; U28.VDDIO_MEM_S3 8,3; U29.VSS 9,3; U30.VDDIO_MEM_S3 10,3; U31.VSS 11,3; U32.VDDIO_MEM_S3 12,3; U33.MA_CLK_H[1] 13,3; U34.MA_CLK_L[0] 14,3; U35.VDDIO_MEM_S3 15,3; U36.MB_ADD[1] 16,3; U37.MB_ADD[2] 17,3; U38.VDDIO_MEM_S3 18,3; U39.MB_CLK_H[0] 19,3; V1.VSS -19,2; V2.P_GFX_TXP[14] -18,2; V3.P_GFX_TXN[13] -17,2; V4.VSS -16,2; V5.P_GFX_RXN[15] -15,2; V6.P_GFX_RXP[15] -14,2; V7.VSS -13,2; V8.P0A_ZVSS -12,2; V9.VDDCR_CPU -11,2; V10.VSS -10,2; V11.VDDCR_CPU -9,2; V12.VSS -8,2; V13.VDDCR_SOC -7,2; V27.VDDIO_MEM_S3 7,2; V28.VSS 8,2; V29.VDDIO_MEM_S3 9,2; V30.VSS 10,2; V31.VDDIO_MEM_S3 11,2; V32.MA_CLK_H[3] 12,2; V33.MA_CLK_L[1] 13,2; V34.VDDIO_MEM_S3 14,2; V35.MA_CLK_H[2] 15,2; V36.MA_CLK_L[2] 16,2; V37.VDDIO_MEM_S3 17,2; V38.MB_CLK_H[1] 18,2; V39.MB_CLK_L[0] 19,2; W1.P_GFX_TXP[15] -19,1; W2.P_GFX_TXN[14] -18,1; W3.VDDCR_CPU -17,1; W4.P_HUB_RXP[3] -16,1; W5.P_HUB_RXN[3] -15,1; W6.VDDCR_CPU -14,1; W7.P_ZVSS -13,1; W8.P_ZVDDP -12,1; W9.VSS -11,1; W10.VDDCR_CPU -10,1; W11.VSS -9,1; W12.VDDCR_CPU -8,1; W13.VSS -7,1; W27.VSS 7,1; W28.VDDIO_MEM_S3 8,1; W29.VSS 9,1; W30.TEST40 10,1; W31.VSS 11,1; W32.MA_CLK_L[3] 12,1; W33.VDDIO_MEM_S3 13,1; W34.VDDIO_MEM_S3 14,1; W35.MA_EVENT_L 15,1; W36.VDDIO_MEM_S3 16,1; W37.MB_CLK_H[2] 17,1; W38.MB_CLK_L[1] 18,1; W39.VDDIO_MEM_S3 19,1; Y1.P_GFX_TXN[15] -19,0; Y2.VDDCR_CPU -18,0; Y3.USB_SS_0RXP -17,0; Y4.USB_SS_0RXN -16,0; Y5.VSS -15,0; Y6.P_HUB_RXP[2] -14,0; Y7.P_HUB_RXN[2] -13,0; Y8.VSS -12,0; Y9.VDDCR_CPU -11,0; Y10.VSS -10,0; Y11.VDDCR_CPU -9,0; Y12.VSS -8,0; Y13.VDDCR_CPU -7,0; Y27.VDDIO_MEM_S3 7,0; Y28.VSS 8,0; Y29.VDDIO_MEM_S3 9,0; Y30.VSS 10,0; Y31.VDDIO_MEM_S3 11,0; Y32.VDDIO_MEM_S3 12,0; Y33.MA_PARTOUT 13,0; Y34.MA__ZVDDIO_MEM_S3 14,0; Y35.VDDIO_MEM_S3 15,0; Y36.MB__ZVDDIO_MEM_S3 16,0; Y37.MB_CLK_L[2] 17,0; Y38.VDDIO_MEM_S3 18,0; Y39.MB_CLK_H[3] 19,0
